(* Logix 5000 AddOnInstructionDefinition export H_ACOMM; software revision 34.01 *)

TYPE HIWIN_MIKRO_AXIS :   // HIWIN MIKROSYSTEM Servo Axis Object
STRUCT
   InData : HIWIN_MIKRO_AXIS_InData;
   OutData : HIWIN_MIKRO_AXIS_OutData;
   ConnectionFaulted : BOOL; {access Read Only}
END_STRUCT
END_TYPE

TYPE HIWIN_MIKRO_AXIS_InData :   // HIWIN MIKROSYSTEM Input Data
STRUCT
   ModesOfOperationDisplay : INT; {access Read Only}   // 6061
   Statusword : INT; {access Read Only}   // 6041
   PositionActualValue : DINT; {access Read Only}   // 6064
   VelocityActualValue : DINT; {access Read Only}   // 606C
   TorqueActualValue : INT; {access Read Only}   // 6077
   Statusword2 : HIWIN_MIKRO_Statusword2; {access None}
   FollowingErrorActualValue : DINT; {access Read Only}   // 60F4
   Rsv1 : INT; {access Read Only}   // Reserve
   DriveAlarmCode : INT; {access Read Only}
   DriveWarningCode : INT; {access Read Only}
   TouchProbeStatus : INT; {access Read Only}   // 60B9
   TouchProbe_1_PositiveEdge : DINT; {access Read Only}   // 60BA
   TouchProbe_2_PositiveEdge : DINT; {access Read Only}   // 60BA
   DigitalInput : DINT; {access Read Only}   // 60FD (bit0: P-OT, bit1: N-OT, bit16~23: I1~I8)
   Rsv2 : INT; {access Read Only}   // Reserve
   Rsv3 : INT; {access Read Only}   // Reserve
   Rsv4 : INT; {access Read Only}   // Reserve
   Rsv5 : INT; {access Read Only}   // Reserve
   UserParmMappingState : DINT; {access Read Only}   // User defined parameter mapping state
   UserMON_1 : DINT; {access Read Only}   // User defined monitor parameter 1
   UserMON_2 : DINT; {access Read Only}   // User defined monitor parameter 2
   UserMON_3 : DINT; {access Read Only}   // User defined monitor parameter 3
END_STRUCT
END_TYPE

TYPE HIWIN_MIKRO_AXIS_OutData :   // HIWIN MIKROSYSTEM Output Data
STRUCT
   ModesOfOperation : INT;   // 6060
   Controlword : INT;   // 6040
   TargetPosition : DINT;   // 607A
   TargetVelocity : DINT;   // 60FF
   TargetTorque : INT;   // 6071
   Controlword2 : INT;
   ProfileVelocity : DINT;   // 6081
   ProfileAcceleration : DINT;   // 6083
   ProfileDeceleration : DINT;   // 6084
   TorqueSlope : DINT;   // 6087
   Rsv1 : INT;   // Reserve
   TouchProbeFunction : INT;   // 60B8
   DigitalOutput : DINT;   // 60FE:01 (bit16~bit19: O1~O4)
   Rsv2 : INT;   // Reserve
   Rsv3 : INT;   // Reserve
   Rsv4 : INT;   // Reserve
   Rsv5 : INT;   // Reserve
   UserParmMappingCtrl : DINT; {access Read Only}   // User defined parameter mapping control
   UserCMD_1 : DINT;   // User defined command parameter 1
   UserCMD_2 : DINT;   // User defined command parameter 2
   UserCMD_3 : DINT;   // User defined command parameter 3
END_STRUCT
END_TYPE

TYPE HIWIN_MIKRO_Statusword2 :   // HIWIN MIKROSYSTEM Statusword2 Bit
STRUCT
   D_RDY : BOOL; {access Read Only}
   S_RDY : BOOL; {access Read Only}
   SF1 : BOOL; {access Read Only}   // STO SF1
   SF2 : BOOL; {access Read Only}   // STO SF2
   STO : BOOL; {access Read Only}   // STO
   BK : BOOL; {access Read Only}   // Brake
   CLT : BOOL; {access Read Only}   // Current Limit Active Status
   VLT : BOOL; {access Read Only}   // Velocity Limit Active Status
   COIN_VCMP : BOOL; {access Read Only}   // COIN/V_CMP Status
   NEAR : BOOL; {access Read Only}
   HOMED : BOOL; {access Read Only}
   INDEX : BOOL; {access Read Only}
   Rsv1 : BOOL; {access Read Only}
   Rsv2 : BOOL; {access Read Only}
   Rsv3 : BOOL; {access Read Only}
   Rsv4 : BOOL; {access Read Only}
END_STRUCT
END_TYPE

ADD_ON_INSTRUCTION H_ACOMM   (* revision 1.2, vendor HIWIN MIKROSYSTEM CORP., ExecutePrescan, ExecuteEnableInFalse *)
// HIWIN MIKROSYSTEM Axis Communication instruction.
// Revision note:
// Check the revision detail in Function Blocks (AOIs) Application Manual.
// Help:
// The H_ACOMM is used for drive motion and parameter IO data transmission. Each HIWIN MIKROSYSTEM axis needs a H_ACOMM instruction to create the transmission channel and remain this instruction always in enable state
VAR_IN_OUT
   InputData : INT[32]; {required}   // module:I.Data Eg. E2:I.Data
   OutputData : INT[32]; {required}   // module:O.Data Eg. E2:O.Data
   H_Axis : HIWIN_MIKRO_AXIS; {required}
END_VAR
VAR_INPUT
   ConnectionFaulted : BOOL; {required}   // 1: In connection fault state
END_VAR
VAR_OUTPUT
   EN : BOOL; {access Read Only, visible}   // 1: Instruction is enabled
   PLCControllable : BOOL; {access Read Only, visible}   // 1: Axis is controllable by PLC
   DrvErr : BOOL; {access Read Only, visible}   // 1: Drive is in alarm state
   DrvErrCode : INT; {access Read Only, visible}   // Drive error code
   DrvWarn : BOOL; {access Read Only, visible}   // 1: Drive is in warning state
   DrvWarnCode : INT; {access Read Only, visible}   // Drive warning code
   InternalLimit : BOOL; {access Read Only}   // 1: A drive internal limit is active
END_VAR
VAR
   SINT_Array : SINT[2]; {access None}
END_VAR

ROUTINE EnableInFalse   (* structured text *)
   
   // Reset output state, data
   EN := 0;
   PLCControllable := 0;
   DrvErr := 0;
   DrvWarn := 0;
   InternalLimit := 0;
   DrvErrCode := 0;
   DrvWarnCode := 0;
   
   
END_ROUTINE

ROUTINE Logic   (* structured text *)
// HIWIN MIKROSYSTEM Axis Communication
   
   //========================================
   // Update input data (drive -> controller)
   //========================================
   H_Axis.InData.ModesOfOperationDisplay	:= InputData[0];
   H_Axis.InData.Statusword				:= InputData[1];
   
   CPS(InputData[2], H_Axis.InData.PositionActualValue, 1);
   CPS(InputData[4], H_Axis.InData.VelocityActualValue, 1);
   
   H_Axis.InData.TorqueActualValue			:= InputData[6];
   
   CPS(InputData[7], H_Axis.InData.Statusword2, 1);
   CPS(InputData[8], H_Axis.InData.FollowingErrorActualValue, 1);
   
   H_Axis.InData.Rsv1 := InputData[10];
   H_Axis.InData.DriveAlarmCode			:= InputData[11];
   H_Axis.InData.DriveWarningCode			:= InputData[12];
   H_Axis.InData.TouchProbeStatus			:= InputData[13];
   
   CPS(InputData[14], H_Axis.InData.TouchProbe_1_PositiveEdge, 1);
   CPS(InputData[16], H_Axis.InData.TouchProbe_2_PositiveEdge, 1);
   CPS(InputData[18], H_Axis.InData.DigitalInput, 1);
   
   H_Axis.InData.Rsv2 := InputData[20];
   H_Axis.InData.Rsv3 := InputData[21];
   H_Axis.InData.Rsv4 := InputData[22];
   H_Axis.InData.Rsv5 := InputData[23];
   
   CPS(InputData[24], H_Axis.InData.UserParmMappingState, 1);
   CPS(InputData[26], H_Axis.InData.UserMON_1, 1);
   CPS(InputData[28], H_Axis.InData.UserMON_2, 1);
   CPS(InputData[30], H_Axis.InData.UserMON_3, 1);
   
   
   //=========================================
   // Update output data (controller -> drive)
   //=========================================
   OutputData[0] := H_Axis.OutData.ModesOfOperation;
   OutputData[1] := H_Axis.OutData.Controlword;
   
   CPS(H_Axis.OutData.TargetPosition, OutputData[2], 2);
   CPS(H_Axis.OutData.TargetVelocity, OutputData[4], 2);
   
   OutputData[6] := H_Axis.OutData.TargetTorque;
   OutputData[7] := H_Axis.OutData.Controlword2;
   
   CPS(H_Axis.OutData.ProfileVelocity, OutputData[8], 2);
   CPS(H_Axis.OutData.ProfileAcceleration, OutputData[10], 2);
   CPS(H_Axis.OutData.ProfileDeceleration, OutputData[12], 2);
   CPS(H_Axis.OutData.TorqueSlope, OutputData[14], 2);
   
   OutputData[16] := H_Axis.OutData.Rsv1;
   OutputData[17] := H_Axis.OutData.TouchProbeFunction;
   
   CPS(H_Axis.OutData.DigitalOutput, OutputData[18], 2);
   OutputData[20] := H_Axis.OutData.Rsv2;
   OutputData[21] := H_Axis.OutData.Rsv3;
   OutputData[22] := H_Axis.OutData.Rsv4;
   OutputData[23] := H_Axis.OutData.Rsv5;
   
   CPS(H_Axis.OutData.UserParmMappingCtrl, OutputData[24], 2);
   CPS(H_Axis.OutData.UserCMD_1, OutputData[26], 2);
   CPS(H_Axis.OutData.UserCMD_2, OutputData[28], 2);
   CPS(H_Axis.OutData.UserCMD_3, OutputData[30], 2);
   
   
   // Update PLCControllable state
   PLCControllable := H_Axis.InData.Statusword.9;
   
   // Update drive error state
   DrvErr := ConnectionFaulted OR H_Axis.InData.Statusword.3;
   
   // Update drive error code
   if DrvErr then
   	DrvErrCode := H_Axis.InData.DriveAlarmCode;
   else
   	DrvErrCode := 0;
   end_if;
   
   // Update drive warning state
   DrvWarn := H_Axis.InData.Statusword.7;
   
   // Update drive warning code
   if DrvWarn then
   	DrvWarnCode := H_Axis.InData.DriveWarningCode;
   else
   	DrvWarnCode := 0;
   end_if;
   
   // Update Internal Limit state
   InternalLimit := H_Axis.InData.Statusword.11;
   
   // Connection Fault
   H_Axis.ConnectionFaulted := ConnectionFaulted;
   
   // Shutdown Condition
   if (H_Axis.ConnectionFaulted
   	OR H_Axis.InData.Statusword.3
   	OR NOT PLCControllable
   	) then
   	// set Shutdown
   	H_Axis.OutData.Controlword.0 := 0;
   	H_Axis.OutData.Controlword.1 := 1;
   	H_Axis.OutData.Controlword.2 := 1;
   	H_Axis.OutData.Controlword.3 := 0;
   end_if;
   
   EN := EnableOut;
   
END_ROUTINE

ROUTINE Prescan   (* structured text *)
   // Initialize variables
   SINT_Array[0] := 0;
   SINT_Array[1] := 0;
   
   COP(SINT_Array[0] ,InputData[0], 32);
   COP(SINT_Array[0] ,OutputData[0], 32);
   
   H_Axis.InData.ModesOfOperationDisplay := 0;
   H_Axis.InData.Statusword := 0;
   H_Axis.InData.PositionActualValue := 0;
   H_Axis.InData.VelocityActualValue := 0;
   H_Axis.InData.TorqueActualValue := 0;
   COP(SINT_Array[0], H_Axis.InData.Statusword2, 1);
   H_Axis.InData.FollowingErrorActualValue := 0;
   H_Axis.InData.DigitalInput := 0;
   H_Axis.InData.DriveAlarmCode := 0;
   H_Axis.InData.DriveWarningCode := 0;
   H_Axis.InData.TouchProbeStatus := 0;
   H_Axis.InData.TouchProbe_1_PositiveEdge := 0;
   H_Axis.InData.TouchProbe_2_PositiveEdge := 0;
   H_Axis.InData.Rsv2 := 0;
   H_Axis.InData.Rsv3 := 0;
   H_Axis.InData.Rsv4 := 0;
   H_Axis.InData.Rsv5 := 0;
   H_Axis.InData.UserParmMappingState := 0;
   H_Axis.InData.UserMON_1 := 0;
   H_Axis.InData.UserMON_2 := 0;
   H_Axis.InData.UserMON_3 := 0;
   
   
   H_Axis.OutData.ModesOfOperation := 0;
   H_Axis.OutData.Controlword := 6;
   H_Axis.OutData.TargetPosition := 0;
   H_Axis.OutData.TargetVelocity := 0;
   H_Axis.OutData.TargetTorque := 0;
   H_Axis.OutData.Controlword2 := 0;
   H_Axis.OutData.ProfileVelocity := 0;
   H_Axis.OutData.ProfileAcceleration := 0;
   H_Axis.OutData.ProfileDeceleration := 0;
   H_Axis.OutData.TorqueSlope := 0;
   H_Axis.OutData.DigitalOutput := 0;
   H_Axis.OutData.TouchProbeFunction := 0;
   H_Axis.OutData.Rsv2 := 0;
   H_Axis.OutData.Rsv3 := 0;
   H_Axis.OutData.Rsv4 := 0;
   H_Axis.OutData.Rsv5 := 0;
   H_Axis.OutData.UserParmMappingCtrl := 0;
   H_Axis.OutData.UserCMD_1 := 0;
   H_Axis.OutData.UserCMD_2 := 0;
   H_Axis.OutData.UserCMD_3 := 0;
   
   H_Axis.ConnectionFaulted := 0;
   
   // Init input state, data
   ConnectionFaulted := 0;
   
   // Init output state, data
   EN := 0;
   DrvErr := 0;
   DrvWarn := 0;
   InternalLimit := 0;
   DrvErrCode := 0;
   DrvWarnCode := 0;
   
   
END_ROUTINE
END_ADD_ON_INSTRUCTION

ADD_ON_INSTRUCTION H_AStatus   (* revision 1.1, vendor HIWIN MIKROSYSTEM CORP., ExecutePrescan *)
// HIWIN MIKROSYSTEM Axis Statues instruction.
// Revision note:
// Check the revision detail in Function Blocks (AOIs) Application Manual.
VAR_IN_OUT
   H_Axis : HIWIN_MIKRO_AXIS; {required}
END_VAR
VAR_OUTPUT
   EN : BOOL; {access Read Only, visible}   // 1: Instruction is enabled
   DrvWarnCode : INT; {access Read Only, visible}   // Drive warning code
   DrvErrCode : INT; {access Read Only, visible}   // Drive error code
   D_RDY : BOOL; {access Read Only, visible}   // Drive Ready state
   S_RDY : BOOL; {access Read Only, visible}   // Servo Ready state
   DrvErr : BOOL; {access Read Only, visible}   // Drive error status
   DrvWarn : BOOL; {access Read Only, visible}   // Drive warning status
   STO : BOOL; {access Read Only, visible}   // STO active state
   SF1 : BOOL; {access Read Only, visible}   // STO SF1 input state
   SF2 : BOOL; {access Read Only, visible}   // STO SF2 input state
   BK : BOOL; {access Read Only, visible}   // Brake active state
   CLT : BOOL; {access Read Only, visible}   // Torque limit detection state
   VLT : BOOL; {access Read Only, visible}   // Velocity limit detection state
   COIN : BOOL; {access Read Only, visible}   // Positioning completion state
   V_CMP : BOOL; {access Read Only, visible}   // Velocity reach state
   NEAR : BOOL; {access Read Only, visible}   // Positioning near state
   HOMED : BOOL; {access Read Only, visible}   // Homing state
   INDEX : BOOL; {access Read Only, visible}   // Index signal output
   P_OT : BOOL; {access Read Only, visible}   // Positive limit switch
   N_OT : BOOL; {access Read Only, visible}   // Negative limit switch
   HomeSwitch : BOOL; {access Read Only, visible}   // Home switch (DOG)
   I1 : BOOL; {access Read Only, visible}   // Digital input status
   I2 : BOOL; {access Read Only, visible}   // Digital input status
   I3 : BOOL; {access Read Only, visible}   // Digital input status
   I4 : BOOL; {access Read Only, visible}   // Digital input status
   I5 : BOOL; {access Read Only, visible}   // Digital input status
   I6 : BOOL; {access Read Only, visible}   // Digital input status
   I7 : BOOL; {access Read Only, visible}   // Digital input status
   I8 : BOOL; {access Read Only, visible}   // Digital input status
END_VAR

ROUTINE Logic   (* structured text *)
// HIWIN MIKROSYSTEM Axis Servo ON
   
   D_RDY := H_Axis.InData.Statusword2.D_RDY;
   S_RDY := H_Axis.InData.Statusword2.S_RDY;
   SF1 := H_Axis.InData.Statusword2.SF1;
   SF2 := H_Axis.InData.Statusword2.SF2;
   STO := H_Axis.InData.Statusword2.STO;
   BK := H_Axis.InData.Statusword2.BK;
   CLT := H_Axis.InData.Statusword2.CLT;
   VLT := H_Axis.InData.Statusword2.VLT;
   COIN := H_Axis.InData.Statusword2.COIN_VCMP;
   V_CMP := H_Axis.InData.Statusword2.COIN_VCMP;
   NEAR := H_Axis.InData.Statusword2.NEAR;
   HOMED := H_Axis.InData.Statusword2.HOMED;
   INDEX := H_Axis.InData.Statusword2.INDEX;
   
   DrvErr := H_Axis.InData.Statusword.3;
   DrvWarn := H_Axis.InData.Statusword.7;
   
   // Update drive error code
   if DrvErr then
   	DrvErrCode := H_Axis.InData.DriveAlarmCode;
   else
   	DrvErrCode := 0;
   end_if;
   
   // Update drive warning code
   if DrvWarn then
   	DrvWarnCode := H_Axis.InData.DriveWarningCode;
   else
   	DrvWarnCode := 0;
   end_if;
   
   P_OT := H_Axis.InData.DigitalInput.0;
   N_OT := H_Axis.InData.DigitalInput.1;
   
   I1 := H_Axis.InData.DigitalInput.16;
   I2 := H_Axis.InData.DigitalInput.17;
   I3 := H_Axis.InData.DigitalInput.18;
   I4 := H_Axis.InData.DigitalInput.19;
   I5 := H_Axis.InData.DigitalInput.20;
   I6 := H_Axis.InData.DigitalInput.21;
   I7 := H_Axis.InData.DigitalInput.22;
   I8 := H_Axis.InData.DigitalInput.23;
   
END_ROUTINE

ROUTINE Prescan   (* structured text *)
   
   // Init output state, data
   EN := 0;
   
   D_RDY := 0;
   S_RDY := 0;
   SF1 := 0;
   SF2 := 0;
   STO := 0;
   BK := 0;
   CLT := 0;
   VLT := 0;
   COIN := 0;
   V_CMP := 0;
   NEAR := 0;
   HOMED := 0;
   INDEX := 0;
   
   I1 := H_Axis.InData.DigitalInput.16;
   I2 := H_Axis.InData.DigitalInput.17;
   I3 := H_Axis.InData.DigitalInput.18;
   I4 := H_Axis.InData.DigitalInput.19;
   I5 := H_Axis.InData.DigitalInput.20;
   I6 := H_Axis.InData.DigitalInput.21;
   I7 := H_Axis.InData.DigitalInput.22;
   I8 := H_Axis.InData.DigitalInput.23;
   
END_ROUTINE
END_ADD_ON_INSTRUCTION

ADD_ON_INSTRUCTION H_MAFR   (* revision 1.1, vendor HIWIN MIKROSYSTEM CORP., ExecutePrescan, ExecuteEnableInFalse *)
// HIWIN MIKROSYSTEM Axis Alarm Reset instruction.
// Revision note:
// Check the revision detail in Function Blocks (AOIs) Application Manual.
// Help:
// The H_MAFR is used to clear the drive alarms of a HIWIN MIKROSYSTEM axis.
// The command needs 20ms for execution. After 20ms, the fault reset command of Controlword will be cleared and the output of .PC will shows if drive alarms are reset successfully.
// This instruction is executed at the rising edge of enabling.
VAR_IN_OUT
   H_Axis : HIWIN_MIKRO_AXIS; {required}
END_VAR
VAR_OUTPUT
   EN : BOOL; {access Read Only, visible}   // 1: Instruction is enabled
   DN : BOOL; {access Read Only, visible}   // 1: Command execution is done
   PC : BOOL; {access None, visible}   // 1: Faults reset successfully
   IP : BOOL; {access None, visible}   // 1: Command is in processing
END_VAR
VAR
   dbOSRI : FBD_ONESHOT; {access None}
   TONR_waitToCheckState : FBD_TIMER; {access None}
   dbOSFI : FBD_ONESHOT; {access None}
END_VAR

ROUTINE EnableInFalse   (* structured text *)
   
   // Reset input
   EN := 0;
   
   // Rest OSRI func
   dbOSRI.InputBit := EnableIn;
   OSRI(dbOSRI);
   
   dbOSFI.InputBit := EnableIn;
   OSFI(dbOSFI);
   
   if dbOSFI.OutputBit then
   	TONR_waitToCheckState.PRE := 20 - TONR_waitToCheckState.ACC;
   end_if;
   
   if IP AND NOT DN then
   	TONR_waitToCheckState.TimerEnable := 1;
   	TONR(TONR_waitToCheckState);
   
   	if TONR_waitToCheckState.DN then
   		TONR_waitToCheckState.TimerEnable := 0;
   		TONR(TONR_waitToCheckState);
   		IP := 0;
   		DN := 1;
   	end_if;
   end_if;
   
   if NOT IP AND DN then
   	H_Axis.OutData.Controlword.7 := 0;
   	if NOT ((H_Axis.InData.Statusword & 16#0008) = 16#0008) then
   		PC := 1;
   	end_if;
   end_if;
   
   
   
END_ROUTINE

ROUTINE Logic   (* structured text *)
// HIWIN MIKROSYSTEM Axis Fault Reset
   // detact rising edge enable signal
   dbOSRI.InputBit := EnableIn;
   OSRI(dbOSRI);
   
   dbOSFI.InputBit := EnableIn;
   OSFI(dbOSFI);
   
   if dbOSRI.OutputBit then
   	H_Axis.OutData.Controlword.7 := 1;
   	IP := 1;
   	DN := 0;
   	PC := 0;
   end_if;
   
   if IP AND NOT DN then
   	TONR_waitToCheckState.PRE := 20; // 20ms delay
   	TONR_waitToCheckState.TimerEnable := 1;
   	TONR(TONR_waitToCheckState);
   
   	if TONR_waitToCheckState.DN then
   		TONR_waitToCheckState.TimerEnable := 0;
   		TONR(TONR_waitToCheckState);
   		IP := 0;
   		DN := 1;
   	end_if;
   end_if;
   
   if NOT IP AND DN then
   	H_Axis.OutData.Controlword.7 := 0;
   	if NOT ((H_Axis.InData.Statusword & 16#0008) = 16#0008) then
   		PC := 1;
   	end_if;
   end_if;
   
   EN := EnableOut;
   
   
END_ROUTINE

ROUTINE Prescan   (* structured text *)
   
   // Init output state, data
   EN := 0;
   DN := 0;
   
   // Init OSRI func
   dbOSRI.InputBit := 0;
   OSRI(dbOSRI);
   
   dbOSFI.InputBit := 0;
   OSFI(dbOSFI);
   
   // Reset H_Axis output data
   H_Axis.OutData.Controlword.7 := 0;
   
END_ROUTINE
END_ADD_ON_INSTRUCTION

ADD_ON_INSTRUCTION H_MAH   (* revision 1.2, vendor HIWIN MIKROSYSTEM CORP., ExecutePrescan, ExecuteEnableInFalse *)
// HIWIN MIKROSYSTEM Axis Homing instruction
// Revision note:
// Check the revision detail in Function Blocks (AOIs) Application Manual.
// Help:
// The H_MAH is used to start a CiA402 homing process on a HIWIN MIKROSYSTEM axis. The information of supported home methods is described at the drive EtherNet/IP communication command manual. (eg, E2 Series Servo Drive EtherNet_IP Communication Command Manual)
// This instruction is executed at the rising edge of enabling.
// To stop a homing process, call the H_MAS to cancel an executing command.
// [Input parameters unit]
// SearchSwitchSpeed: control unit
// SearchZeroPoint: control unit
// HomeOffset:  control unit
// [Instruction Error Codes]
// -1: PLC not controllable
// -2: Drive is in alarm state
// -3: Drive not ready
// -4: Servo not ready
// -5: Homing fail
// others: The MSG instruction error codes (referring to the Logix 5000 instruction Help file)
VAR_IN_OUT
   H_Axis : HIWIN_MIKRO_AXIS; {required}
END_VAR
VAR_INPUT
   Method : DINT; {access None, required}   // CiA402 homing method
   SearchSwitchSpeed : DINT; {access None, required}   // Calibration point (eg, a limit switch or a near home sensor) searching speed
   SearchZeroSpeed : DINT; {access None, required}   // Home point searching speed
   Acceleration : DINT; {access None, required}   // Homing acceleration
   HomeOffset : DINT; {access None, required}   // Home offset value
END_VAR
VAR_OUTPUT
   EN : BOOL; {access Read Only, visible}   // 1: Instruction is enabled
   DN : BOOL; {access Read Only, visible}   // 1: Homing process is completed or aborted
   IP : BOOL; {access Read Only, visible}   // 1: Homing process is busy
   PC : BOOL; {access Read Only, visible}   // 1: Homing is successfully completed
   ER : BOOL; {access Read Only, visible}   // 1: Instruction detect an error
   ErrCode : INT; {access Read Only, visible}   // Instruction error code
END_VAR
VAR_IN_OUT
   HomeMsgWriteCtrl : MESSAGE; {required}   // Message read/write object struct
END_VAR
VAR_INPUT
   MsgWriteData : DINT; {access None}   // DO NOT CHANGE (used to set the HomeMsgWriteCtrl 'source element')
END_VAR
VAR
   dbOSRI : FBD_ONESHOT; {access None}
   LocalStepCtrl : DINT; {access None}
   dbOSFI : FBD_ONESHOT; {access None}
   OSFI_IP : FBD_ONESHOT; {access None}
   TONR_waitToCheckState : FBD_TIMER; {access None}
END_VAR

ROUTINE EnableInFalse   (* structured text *)
   
   // Reset output state, data
   EN := 0;
   
   // Rest OSRI func
   dbOSRI.InputBit := EnableIn;
   OSRI(dbOSRI);
   
   dbOSFI.InputBit := EnableIn;
   OSFI(dbOSFI);
   
   if dbOSFI.OutputBit then
   	TONR_waitToCheckState.PRE := 50 - TONR_waitToCheckState.ACC;
   end_if;
   
   OSFI_IP.InputBit := IP;
   OSFI(OSFI_IP);
   if OSFI_IP.OutputBit then
   	H_Axis.OutData.Controlword.4 := 0;
   	OSFI_IP.InputBit := 0;
   	OSFI(OSFI_IP);
   end_if;
   
   if (LocalStepCtrl > 5) then
   
   	TONR_waitToCheckState.TimerEnable := 1;
   	TONR(TONR_waitToCheckState);
   
   	if TONR_waitToCheckState.DN then
   		if (H_Axis.InData.ModesOfOperationDisplay = 6) then
   			if H_Axis.InData.Statusword.13 then
   				// home error
   				IP := 0;
   				DN := 1;
   				ER := 1;
   				ErrCode := -5; // home fail
   				LocalStepCtrl := 0;
   
   			elsif H_Axis.InData.Statusword.10 & H_Axis.InData.Statusword.12 then
   				// home success and complete
   				IP := 0;
   				DN := 1;
   				PC := 1;
   				LocalStepCtrl := 0;
   
   			elsif H_Axis.InData.Statusword.10 & NOT H_Axis.InData.Statusword.12 & NOT H_Axis.OutData.Controlword.4 then
   				// homing process is stopped by H_MAS
   				IP := 0;
   				DN := 1;
   				PC := 0;
   				LocalStepCtrl := 0;
   
   			end_if;
   		else
   			if IP & NOT DN then
   				IP := 0;
   				DN := 1;
   				ER := 1;
   				ErrCode := -5; // home fail
   				LocalStepCtrl := 0;
   			end_if;
   		end_if;
   	end_if;
   else
   	if IP & NOT DN then
   		IP := 0;
   		DN := 1;
   		LocalStepCtrl := 0;
   	end_if;
   end_if;
   
   if NOT IP & DN then
   	TONR_waitToCheckState.TimerEnable := 0;
   	TONR(TONR_waitToCheckState);
   end_if;
   
   
   
END_ROUTINE

ROUTINE Logic   (* structured text *)
// HIWIN MIKROSYSTEM Motion Axis Homing
   
   // detact rising edge enable signal
   dbOSRI.InputBit := EnableIn;
   OSRI(dbOSRI);
   
   dbOSFI.InputBit := EnableIn;
   OSFI(dbOSFI);
   
   if dbOSRI.OutputBit then
   	IP := 1;
   	DN := 0;
   	ER := 0;
   	PC := 0;
   	ErrCode := 0;
   
   	//Request mode change
   	H_Axis.OutData.ModesOfOperation := 6; // set to Home mode
   	H_Axis.OutData.Controlword.4 := 0; // clear home start bit
   
   	LocalStepCtrl := 0;
   end_if;
   
   if IP & NOT DN then
   	if NOT H_Axis.InData.Statusword.9 then
   		IP := 0;
   		DN := 1;
   		ER := 1;
   		ErrCode := -1; // PLC not Controllable
   	elsif H_Axis.InData.Statusword.3 then
   		IP := 0;
   		DN := 1;
   		ER := 1;
   		ErrCode := -2; // Drive alarm
   	elsif NOT H_Axis.InData.Statusword2.D_RDY then
   		IP := 0;
   		DN := 1;
   		ER := 1;
   		ErrCode := -3; // Drive not ready
   	elsif NOT H_Axis.InData.Statusword2.S_RDY then
   		IP := 0;
   		DN := 1;
   		ER := 1;
   		ErrCode := -4; // Servo not ready
   	else
   		case LocalStepCtrl of
   			0: // write home method (0x6098)
   				HomeMsgWriteCtrl.Class := 16#406;
   				HomeMsgWriteCtrl.Instance := 16#098;
   				HomeMsgWriteCtrl.Attribute := 0;
   				HomeMsgWriteCtrl.REQ_LEN := 1;
   				MsgWriteData := Method;
   				MSG(HomeMsgWriteCtrl);
   
   				LocalStepCtrl := LocalStepCtrl + 1;
   
   			1: // write home acceleration (0x609A)
   				//check parameter write status
   				if NOT HomeMsgWriteCtrl.ER then
   					if HomeMsgWriteCtrl.DN then
   
   						HomeMsgWriteCtrl.Class := 16#406;
   						HomeMsgWriteCtrl.Instance := 16#09A;
   						HomeMsgWriteCtrl.Attribute := 0;
   						HomeMsgWriteCtrl.REQ_LEN := 4;
   						MsgWriteData := Acceleration;
   						MSG(HomeMsgWriteCtrl);
   
   						LocalStepCtrl := LocalStepCtrl + 1;
   					end_if;
   				else
   					IP := 0;
   					DN := 1;
   					ER := 1;
   					ErrCode := HomeMsgWriteCtrl.ERR;
   				end_if;
   
   			2: // write search switch speed (0x6099_01)
   				//check parameter write status
   				if NOT HomeMsgWriteCtrl.ER then
   					if HomeMsgWriteCtrl.DN then
   
   						HomeMsgWriteCtrl.Class := 16#406;
   						HomeMsgWriteCtrl.Instance := 16#099;
   						HomeMsgWriteCtrl.Attribute := 1;
   						HomeMsgWriteCtrl.REQ_LEN := 4;
   						MsgWriteData := SearchSwitchSpeed;
   						MSG(HomeMsgWriteCtrl);
   
   						LocalStepCtrl := LocalStepCtrl + 1;
   					end_if;
   				else
   					IP := 0;
   					DN := 1;
   					ER := 1;
   					ErrCode := HomeMsgWriteCtrl.ERR;
   				end_if;
   
   			3: // write search zero speed (0x6099_02)
   				//check parameter write status
   				if NOT HomeMsgWriteCtrl.ER then
   					if HomeMsgWriteCtrl.DN then
   
   						HomeMsgWriteCtrl.Class := 16#406;
   						HomeMsgWriteCtrl.Instance := 16#099;
   						HomeMsgWriteCtrl.Attribute := 2;
   						HomeMsgWriteCtrl.REQ_LEN := 4;
   						MsgWriteData := SearchZeroSpeed;
   						MSG(HomeMsgWriteCtrl);
   
   						LocalStepCtrl := LocalStepCtrl + 1;
   					end_if;
   				else
   					IP := 0;
   					DN := 1;
   					ER := 1;
   					ErrCode := HomeMsgWriteCtrl.ERR;
   				end_if;
   
   			4: // write home offset (0x607C)
   				//check parameter write status
   				if NOT HomeMsgWriteCtrl.ER then
   					if HomeMsgWriteCtrl.DN then
   
   						HomeMsgWriteCtrl.Class := 16#406;
   						HomeMsgWriteCtrl.Instance := 16#07C;
   						HomeMsgWriteCtrl.Attribute := 0;
   						HomeMsgWriteCtrl.REQ_LEN := 4;
   						MsgWriteData := HomeOffset;
   						MSG(HomeMsgWriteCtrl);
   
   						LocalStepCtrl := LocalStepCtrl + 1;
   					end_if;
   				else
   					IP := 0;
   					DN := 1;
   					ER := 1;
   					ErrCode := HomeMsgWriteCtrl.ERR;
   				end_if;
   
   			5:
   				//check parameter write status
   				if NOT HomeMsgWriteCtrl.ER then
   					if HomeMsgWriteCtrl.DN then
   						if (H_Axis.InData.ModesOfOperationDisplay = 6) then
   							// start homing
   							H_Axis.OutData.Controlword.4 := 1;
   							H_Axis.OutData.Controlword.8 := 0;
   
   							LocalStepCtrl := LocalStepCtrl + 1;
   						end_if;
   					end_if;
   				else
   					IP := 0;
   					DN := 1;
   					ER := 1;
   					ErrCode := HomeMsgWriteCtrl.ERR;
   				end_if;
   
   			6:
   				TONR_waitToCheckState.PRE := 50; // 50ms delay
   				TONR_waitToCheckState.TimerEnable := 1;
   				TONR(TONR_waitToCheckState);
   
   				if TONR_waitToCheckState.DN then
   					TONR_waitToCheckState.TimerEnable := 0;
   					TONR(TONR_waitToCheckState);
   					LocalStepCtrl := LocalStepCtrl + 1;
   				end_if;
   			7:
   				if (H_Axis.InData.ModesOfOperationDisplay = 6) then
   					if H_Axis.InData.Statusword.13 then
   						// home error
   						IP := 0;
   						DN := 1;
   						ER := 1;
   						ErrCode := -5; // home fail
   						LocalStepCtrl := 0;
   					elsif H_Axis.InData.Statusword.10 & H_Axis.InData.Statusword.12 then
   						// home success and complete
   						IP := 0;
   						DN := 1;
   						PC := 1;
   						LocalStepCtrl := 0;
   					elsif H_Axis.InData.Statusword.10 & NOT H_Axis.InData.Statusword.12 & NOT H_Axis.OutData.Controlword.4 then
   						// homing process is stopped by H_MAS
   						IP := 0;
   						DN := 1;
   						PC := 0;
   						LocalStepCtrl := 0;
   					end_if;
   				else
   					if IP & NOT DN then
   						IP := 0;
   						DN := 1;
   						ER := 1;
   						ErrCode := -5; // home fail
   						LocalStepCtrl := 0;
   					end_if;
   				end_if;
   		end_case;
   	end_if;
   end_if;
   
   OSFI_IP.InputBit := IP;
   OSFI(OSFI_IP);
   if OSFI_IP.OutputBit then
   	H_Axis.OutData.Controlword.4 := 0;
   	OSFI_IP.InputBit := 0;
   	OSFI(OSFI_IP);
   end_if;
   
   EN := EnableOut;
   
   
END_ROUTINE

ROUTINE Prescan   (* structured text *)
   
   // Init output state, data
   EN := 0;
   IP := 0;
   DN := 0;
   ER := 0;
   PC := 0;
   ErrCode := 0;
   
   // Init OSRI func
   dbOSRI.InputBit := 0;
   OSRI(dbOSRI);
   
   dbOSFI.InputBit := 0;
   OSFI(dbOSFI);
   
   
END_ROUTINE
END_ADD_ON_INSTRUCTION

ADD_ON_INSTRUCTION H_MAJ   (* revision 1.1, vendor HIWIN MIKROSYSTEM CORP., ExecutePrescan, ExecuteEnableInFalse *)
// HIWIN MIKROSYSTEM Axis Jog instruction
// Revision note:
// Check the revision detail in Function Blocks (AOIs) Application Manual.
// Help:
// The H_MAJ is used to an endless jogging of a HIWIN MIKROSYSTEM axis.
// This instruction is executed at the rising edge of enabling.
// A jogging can be stopped by calling H_MAS.
// [Input parameters unit]
// Speed: control unit
// Acceleration: control unit
// Deceleration:  control unit
// [Instruction Error Codes]
// -1: PLC not controllable
// -2: Drive is in alarm state
// -3: Drive not ready
// -4: Servo not ready
VAR_IN_OUT
   H_Axis : HIWIN_MIKRO_AXIS; {required}
END_VAR
VAR_INPUT
   Speed : DINT; {access None, required}   // Jogging speed
   Acceleration : DINT; {access None, required}   // Jogging acceleration
   Deceleration : DINT; {access None, required}   // Jogging deceleration
   Direction : BOOL; {access None, required}   // 0: Forward; 1: Reverse
END_VAR
VAR_OUTPUT
   EN : BOOL; {access Read Only, visible}   // 1: Instruction is enabled
   DN : BOOL; {access Read Only, visible}   // 1: Command is executed
   IP : BOOL; {access Read Only, visible}   // 0: Jogging command is stopped; 1: Jogging command is in execution
   ER : BOOL; {access Read Only, visible}   // 1: Instruction detect an error
   ErrCode : INT; {access Read Only, visible}   // Instruction error code
END_VAR
VAR
   dbOSRI : FBD_ONESHOT; {access None}
END_VAR

ROUTINE EnableInFalse   (* structured text *)
   
   // Reset output state, data
   EN := 0;
   
   // Rest OSRI func
   dbOSRI.InputBit := EnableIn;
   OSRI(dbOSRI);
   
   if NOT H_Axis.InData.Statusword2.S_RDY
   	OR NOT H_Axis.InData.Statusword2.D_RDY
   	OR H_Axis.OutData.Controlword.8  // Halt request
   	then
   	IP := 0;
   
   	H_Axis.OutData.TargetVelocity := 0;
   
   end_if;
   
END_ROUTINE

ROUTINE Logic   (* structured text *)
// HIWIN MIKROSYSTEM Axis Jog
   
   // detact rising edge enable signal
   dbOSRI.InputBit := EnableIn;
   OSRI(dbOSRI);
   
   if dbOSRI.OutputBit then
   	IP := 1;
   	DN := 0;
   	ER := 0;
   	ErrCode := 0;
   
   end_if;
   
   if IP & NOT DN then
   	if NOT H_Axis.InData.Statusword.9 then
   		ER := 1;
   		ErrCode := -1; // PLC not Controllable
   	elsif H_Axis.InData.Statusword.3 then
   		ER := 1;
   		ErrCode := -2; // Drive alarm
   	elsif NOT H_Axis.InData.Statusword2.D_RDY then
   		ER := 1;
   		ErrCode := -3; // Drive not ready
   	elsif NOT H_Axis.InData.Statusword2.S_RDY then
   		ER := 1;
   		ErrCode := -4; // Servo not ready
   	else
   		//Request mode change
   		H_Axis.OutData.ModesOfOperation := 3; // to PV
   
   	end_if;
   
   	if ER then
   		IP := 0;
   		DN := 0;
   	elsif H_Axis.InData.ModesOfOperationDisplay = 3 then
   		IP := 1;
   		DN := 1;
   
   		H_Axis.OutData.Controlword.8 := 0;
   
   		if Direction then
   			H_Axis.OutData.TargetVelocity := Speed * -1;
   		else
   			H_Axis.OutData.TargetVelocity := Speed;
   		end_if;
   		H_Axis.OutData.ProfileAcceleration := Acceleration;
   		H_Axis.OutData.ProfileDeceleration := Deceleration;
   
   	end_if;
   end_if;
   
   if IP & DN then
   	if NOT H_Axis.InData.Statusword2.S_RDY
   		OR NOT H_Axis.InData.Statusword2.D_RDY
   		OR H_Axis.OutData.Controlword.8  // Halt request
   		then
   		IP := 0;
   
   		H_Axis.OutData.TargetVelocity := 0;
   
   	end_if;
   
   end_if;
   
   EN := EnableOut;
   
   
END_ROUTINE

ROUTINE Prescan   (* structured text *)
   
   // Init output state, data
   EN := 0;
   IP := 0;
   DN := 0;
   ER := 0;
   ErrCode := 0;
   
   // Init OSRI func
   dbOSRI.InputBit := 0;
   OSRI(dbOSRI);
   
END_ROUTINE
END_ADD_ON_INSTRUCTION

ADD_ON_INSTRUCTION H_MAM   (* revision 1.1, vendor HIWIN MIKROSYSTEM CORP., ExecutePrescan, ExecuteEnableInFalse *)
// HIWIN MIKROSYSTEM Axis Positioning instruction
// Revision note:
// Check the revision detail in Function Blocks (AOIs) Application Manual.
// Help:
// The H_MAM is used to do positioning of a HIWIN MIKROSYSTEM axis. When execute the instruction every time, the setting will be active immediately.
// This instruction is executed at the rising edge of enabling.
// [Input parameters unit]
// Position: control unit
// Velocity: control unit
// Acceleration: control unit
// Deceleration:  control unit
// [Instruction Error Codes]
// -1: PLC not controllable
// -2: Drive is in alarm state
// -3: Drive not ready
// -4: Servo not ready
VAR_IN_OUT
   H_Axis : HIWIN_MIKRO_AXIS; {required}
END_VAR
VAR_INPUT
   Position : DINT; {required}   // Set position
   Velocity : DINT; {required}   // Moving velocity
   Acceleration : DINT; {required}   // Moving acceleration
   Deceleration : DINT; {required}   // Moving deceleration
   SetRelativeMove : BOOL; {required}   // 0: Move absolute; 1: Move relative
END_VAR
VAR_OUTPUT
   EN : BOOL; {access Read Only, visible}   // 1: Instruction is enabled
   DN : BOOL; {access Read Only, visible}   // 1: Command is executed
   IP : BOOL; {access Read Only, visible}   // 1: Command is in processing
   PC : BOOL; {access Read Only, visible}   // 1: Motor is in-position
   ER : BOOL; {access Read Only, visible}   // 1: Instruction detect an error
   ErrCode : INT; {access Read Only, visible}   // Instruction error code
END_VAR
VAR
   dbOSRI : FBD_ONESHOT; {access None}
   dbOSFI : FBD_ONESHOT; {access None}
END_VAR

ROUTINE EnableInFalse   (* structured text *)
   
   // Reset output state, data
   EN := 0;
   
   // Rest OSRI func
   dbOSRI.InputBit := EnableIn;
   OSRI(dbOSRI);
   
   dbOSFI.InputBit := EnableIn;
   OSFI(dbOSFI);
   
   if dbOSFI.OutputBit then
   
   	H_Axis.OutData.Controlword.4 := 0;
   	H_Axis.OutData.Controlword.5 := 0;
   
   end_if;
   
   if IP
   	& DN
   	& (H_Axis.InData.ModesOfOperationDisplay = 1)
       then
   
   	PC := H_Axis.InData.Statusword2.COIN_VCMP;
   	if PC then
   		IP := 0;
   	elsif H_Axis.OutData.Controlword.8 then
   		IP := 0;
   	end_if;
   end_if;
   
END_ROUTINE

ROUTINE Logic   (* structured text *)
// HIWIN MIKROSYSTEM Axis Positioning
   
   // detact rising edge enable signal
   dbOSRI.InputBit := EnableIn;
   OSRI(dbOSRI);
   
   dbOSFI.InputBit := EnableIn;
   OSFI(dbOSFI);
   
   if dbOSRI.OutputBit then
   	IP := 1;
   	DN := 0;
   	PC := 0;
   	ER := 0;
   	ErrCode := 0;
   
   	//Request mode change
   	H_Axis.OutData.ModesOfOperation := 1; // set to position mode
   end_if;
   
   if IP & NOT DN then
   	if NOT H_Axis.InData.Statusword.9 then
   		ER := 1;
   		ErrCode := -1; // PLC not Controllable
   	elsif H_Axis.InData.Statusword.3 then
   		ER := 1;
   		ErrCode := -2; // Drive alarm
   	elsif NOT H_Axis.InData.Statusword2.D_RDY then
   		ER := 1;
   		ErrCode := -3; // Drive not ready
   	elsif NOT H_Axis.InData.Statusword2.S_RDY then
   		ER := 1;
   		ErrCode := -4; // Servo not ready
   	else
   		if ER then
   			IP := 0;
   			DN := 0;
   		elsif H_Axis.InData.ModesOfOperationDisplay = 1 then
   
   			H_Axis.OutData.TargetPosition := Position;
   			H_Axis.OutData.Controlword.6 := SetRelativeMove;
   			H_Axis.OutData.ProfileVelocity := Velocity;
   			H_Axis.OutData.ProfileAcceleration := Acceleration;
   			H_Axis.OutData.ProfileDeceleration := Deceleration;
   
   			if NOT H_Axis.InData.Statusword.12 then
   				DN := 1;
   
   				H_Axis.OutData.Controlword.4 := 1;
   				H_Axis.OutData.Controlword.5 := 1; // change immediately
   				H_Axis.OutData.Controlword.8 := 0;
   			else
   				H_Axis.OutData.Controlword.4 := 0; // reset the new setpoint command to reset the statusword setpoint acknowledgement bit
   			end_if;
   		end_if;
   	end_if;
   end_if;
   
   if IP
   	& DN
   	& (H_Axis.InData.ModesOfOperationDisplay = 1)
       & H_Axis.InData.Statusword.12
       then
   
   	PC := H_Axis.InData.Statusword2.COIN_VCMP;
   	if PC then
   		IP := 0;
   	elsif H_Axis.OutData.Controlword.8 then
   		IP := 0;
   	end_if;
   end_if;
   
   EN := EnableOut;
   
   
END_ROUTINE

ROUTINE Prescan   (* structured text *)
   
   // Init output state, data
   EN := 0;
   IP := 0;
   DN := 0;
   PC := 0;
   ER := 0;
   ErrCode := 0;
   
   // Init OSRI func
   dbOSRI.InputBit := 0;
   OSRI(dbOSRI);
   
   dbOSFI.InputBit := 0;
   OSFI(dbOSFI);
   
   
END_ROUTINE
END_ADD_ON_INSTRUCTION

ADD_ON_INSTRUCTION H_MAR   (* revision 1.2, vendor HIWIN MIKROSYSTEM CORP., ExecutePrescan, ExecuteEnableInFalse *)
// HIWIN MIKROSYSTEM Axis Arm Registration instruction
// Revision note:
// Check the revision detail in Function Blocks (AOIs) Application Manual.
// Help:
// The H_MAR is used to arm registration event checking one time for a HIWIN MIKROSYSTEM axis. This function links to the CiA402 touch probe function of the axis.
// When the instruction is called, a registration event is armed based on the selected Registration Input (InputNumber) and the specified Trigger Condition (TriggerEdge). When the Registration Input satisfies the Trigger Condition, the motor position will be latched and stored. The latest latched position will be response at the axis input data (.InData) TouchProbe_1_PositiveEdge (word 14~15) or TouchProbe_2_PositiveEdge (word16~17).
// Use H_MDR to disarm the event checking process.
// [Instruction Error Codes]
// -1: PLC not controllable
// -6: Invalid setting value
VAR_IN_OUT
   H_Axis : HIWIN_MIKRO_AXIS; {required}
END_VAR
VAR_INPUT
   InputNumber : DINT; {access None, required}   // 0: Encoder index, 1: Ext_Probe1, 2: Ext_Probe2
   TriggerEdge : BOOL; {access None, required}   // 0: positive edge, 1: negative edge
END_VAR
VAR_OUTPUT
   EN : BOOL; {access Read Only, visible}   // 1: Instruction is enabled
   DN : BOOL; {access Read Only, visible}   // 1: Command is executed
   IP : BOOL; {access Read Only, visible}   // 1: An event checking is in processing
   PC : BOOL; {access None, visible}   // 1: A registration event occurs
   ER : BOOL; {access Read Only, visible}   // 1: Instruction detect an error
   ErrCode : INT; {access Read Only, visible}   // Instruction error code
END_VAR
VAR
   dbOSRI : FBD_ONESHOT; {access None}
   TPSignal : DINT; {access None}
   TPEdge : BOOL; {access None}
   StepCtrl : INT; {access None}   // Step control
   DrvTPStatus : INT; {access None}
END_VAR

ROUTINE EnableInFalse   (* structured text *)
   
   // Reset output state, data
   EN := 0;
   
   // Rest OSRI func
   dbOSRI.InputBit := EnableIn;
   OSRI(dbOSRI);
   
   if IP & DN & NOT ER then // waiting for the latch complete
   
   	DrvTPStatus := H_Axis.InData.TouchProbeStatus & 16#07;
   	if TPEdge then // negative edge
   		if DrvTPStatus = 16#0005 then
   			PC := 1;
   		end_if;
   	else // positive edge
   		if DrvTPStatus = 16#0003 then
   			PC := 1;
   		end_if;
   	end_if;
   
   	if ((DrvTPStatus & 16#0001) = 0) then // touch probe processing is interrupted
   		IP := 0;
   	end_if;
   
   end_if;
   
   if ER then
   	IP := 0;
   elsif IP & DN & PC then
   	IP := 0;
   elsif IP & NOT DN & StepCtrl = 2 then
   	IP := 0;
   	StepCtrl := 0;
   end_if;
   
   
   
END_ROUTINE

ROUTINE Logic   (* structured text *)
// HIWIN MIKROSYSTEM Axis Motion Arm Registration
   
   // detact rising edge enable signal
   dbOSRI.InputBit := EnableIn;
   OSRI(dbOSRI);
   
   if IP & NOT DN then
   	case StepCtrl of
   		1:
   			H_Axis.OutData.TouchProbeFunction := 16#0001;
   			StepCtrl := 2;
   		2:
   			if (H_Axis.InData.TouchProbeStatus = 16#0001) then
   				StepCtrl := 3;
   			end_if;
   		3:
   			case TPSignal of
   				0: // Encoder index
   					H_Axis.OutData.TouchProbeFunction := 16#0015;
   					DN := 1;
   					StepCtrl := 4;
   				1: // Ext_Probe 1
   					if TPEdge then // negative edge
   						H_Axis.OutData.TouchProbeFunction := 16#0021;
   					else // positive edge
   						H_Axis.OutData.TouchProbeFunction := 16#0011;
   					end_if;
   					DN := 1;
   					StepCtrl := 4;
   				else
   					ER := 1;
   					ErrCode := -6; // Invalid setting value
   			end_case;
   	end_case;
   
   elsif IP & DN then // waiting for the latch complete
   
   	DrvTPStatus := H_Axis.InData.TouchProbeStatus & 16#07;
   	if TPEdge then // negative edge
   		if DrvTPStatus = 16#0005 then
   			PC := 1;
   		end_if;
   	else // positive edge
   		if DrvTPStatus = 16#0003 then
   			PC := 1;
   		end_if;
   	end_if;
   
   	if ((DrvTPStatus & 16#0001) = 0) then
   		IP := 0;
   	end_if;
   end_if;
   
   if dbOSRI.OutputBit then
   	IP := 1;
   	DN := 0;
   	ER := 0;
   	PC := 0;
   	ErrCode := 0;
   
   	StepCtrl := 1;
   	TPSignal := InputNumber;
   	TPEdge := TriggerEdge;
   
   	if NOT H_Axis.InData.Statusword.9 then
   		IP := 0;
   		ER := 1;
   		ErrCode := -1; // PLC not controllable
   	elsif TPSignal > 3 then
   		IP := 0;
   		ER := 1;
   		ErrCode := -6; // Invalid setting value
   	end_if;
   end_if;
   
   if ER then
   	IP := 0;
   elsif IP & DN & PC then
   	IP := 0;
   end_if;
   
   EN := EnableOut;
   
   
END_ROUTINE

ROUTINE Prescan   (* structured text *)
   
   // Init output state, data
   EN := 0;
   IP := 0;
   DN := 0;
   ER := 0;
   PC := 0;
   ErrCode := 0;
   
   // Init OSRI func
   dbOSRI.InputBit := 0;
   OSRI(dbOSRI);
   
   // Init local parameters
   StepCtrl := 0;
   TPSignal := 0;
   TPEdge := 0;
   
END_ROUTINE
END_ADD_ON_INSTRUCTION

ADD_ON_INSTRUCTION H_MAS   (* revision 1.1, vendor HIWIN MIKROSYSTEM CORP., ExecutePrescan, ExecuteEnableInFalse *)
// HIWIN MIKROSYSTEM Axis Stop instruction
// Revision note:
// Check the revision detail in Function Blocks (AOIs) Application Manual.
// Help:
// The H_MAS is used to stop a moving on a HIWIN MIKROSYSTEM axis.
// The output .PC shows if the motor is stopped or not according to the setting window of PC (WindowOf_PC). The default value of the WindowOf_PC is 10. If the WindowOf_PC is not given a suitable value, the .PC state may be incorrect.
// [Input parameter unit]
// WindowOf_PC: In torque mode is 0.1% rate torque. Other modes are control unit.
// [Instruction Error Codes]
// -1: PLC not controllable
VAR_IN_OUT
   H_Axis : HIWIN_MIKRO_AXIS; {required}
END_VAR
VAR_OUTPUT
   EN : BOOL; {access Read Only, visible}   // 1: Instruction is enabled
   DN : BOOL; {access Read Only, visible}   // 1: The stop command is executed
   IP : BOOL; {access Read Only, visible}   // 1: The axis is stopping
   PC : BOOL; {access Read Only, visible}   // 1: The axis is stopped
   ER : BOOL; {access Read Only, visible}   // 1: Instruction detect an error
END_VAR
VAR_INPUT
   WindowOf_PC : DINT := 10; {required}   // The window to judge the PC true state
END_VAR
VAR_OUTPUT
   ErrCode : INT; {access Read Only, visible}   // Instruction error code
END_VAR
VAR
   dbOSRI : FBD_ONESHOT; {access None}
END_VAR

ROUTINE EnableInFalse   (* structured text *)
   
   // Reset output state, data
   EN := 0;
   
   // Rest OSRI func
   dbOSRI.InputBit := EnableIn;
   OSRI(dbOSRI);
   
   if ER then
   	IP := 0;
   end_if;
   
   if IP AND DN then
   	if (H_Axis.InData.ModesOfOperationDisplay = 4) then
   		if (ABS(H_Axis.InData.TorqueActualValue) <= WindowOf_PC) then
   			IP := 0;
   			PC := 1;
   		end_if;
   	else
   		if (ABS(H_Axis.InData.VelocityActualValue) <= WindowOf_PC) then
   			IP := 0;
   			PC := 1;
   		end_if;
   	end_if;
   end_if;
   
   
END_ROUTINE

ROUTINE Logic   (* structured text *)
// HIWIN MIKROSYSTEM Motion Axis Stop
   
   // detact rising edge enable signal
   dbOSRI.InputBit := EnableIn;
   OSRI(dbOSRI);
   
   if dbOSRI.OutputBit then
   	IP := 1;
   	DN := 0;
   	PC := 0;
   	ER := 0;
   	ErrCode := 0;
   
   end_if;
   
   if IP & NOT DN then
   	DN := 1;
   
   	if NOT H_Axis.InData.Statusword.9 then
   		IP := 0;
   		ER := 1;
   		ErrCode := -1; // PLC not Controllable
   	else
   		// set Halt to stop motion
   		H_Axis.OutData.Controlword.4 := 0;
   		H_Axis.OutData.Controlword.8 := 1;
   	end_if;
   end_if;
   
   if IP AND DN then
   	if (H_Axis.InData.ModesOfOperationDisplay = 4) then
   		if (ABS(H_Axis.InData.TorqueActualValue) <= WindowOf_PC) then
   			IP := 0;
   			PC := 1;
   		end_if;
   	else
   		if (ABS(H_Axis.InData.VelocityActualValue) <= WindowOf_PC) then
   			IP := 0;
   			PC := 1;
   		end_if;
   	end_if;
   end_if;
   
   EN := EnableOut;
   
   
END_ROUTINE

ROUTINE Prescan   (* structured text *)
   
   // Init output state, data
   EN := 0;
   IP := 0;
   DN := 0;
   PC := 0;
   ER := 0;
   ErrCode := 0;
   
   // Init OSRI func
   dbOSRI.InputBit := 0;
   OSRI(dbOSRI);
   
   
END_ROUTINE
END_ADD_ON_INSTRUCTION

ADD_ON_INSTRUCTION H_MASD   (* revision 1.1, vendor HIWIN MIKROSYSTEM CORP., ExecutePrescan, ExecuteEnableInFalse *)
// HIWIN MIKROSYSTEM Axis Shutdown instruction.
// Revision note:
// Check the revision detail in Function Blocks (AOIs) Application Manual.
// Help:
// The H_MASD is used to make a HIWIN MIKROSYSTEM axis goes into the shutdown state.
// The axis remains in the shutdown state until the H_MASR is executed.
// [Instruction Error Codes]
// -1: PLC not controllable
VAR_IN_OUT
   H_Axis : HIWIN_MIKRO_AXIS; {required}
END_VAR
VAR_OUTPUT
   EN : BOOL; {access Read Only, visible}   // 1: Instruction is enabled
   DN : BOOL; {access Read Only, visible}   // 1: Axis is shutdown successfully
   IP : BOOL; {access Read Only, visible}   // 1: Command is in processing
   ER : BOOL; {access Read Only, visible}   // 1: Instruction detect an error
   ErrCode : INT; {access Read Only, visible}   // Instruction error code
END_VAR
VAR
   dbOSRI : FBD_ONESHOT; {access None}
END_VAR

ROUTINE EnableInFalse   (* structured text *)
   
   // Reset output state, data
   EN := 0;
   
   // Rest OSRI func
   dbOSRI.InputBit := EnableIn;
   OSRI(dbOSRI);
   
   if IP then
   	// check Switch on disable state
   	if H_Axis.InData.Statusword.9 // PLCControllable
   		& NOT H_Axis.InData.Statusword.0  // not switch on
   		& NOT H_Axis.InData.Statusword.1  // not switch on
   		& NOT H_Axis.InData.Statusword.2  // not operation enable
   		& H_Axis.InData.Statusword.6  // switch on disable
   		then
   		IP := 0;
   		DN := 1;
   	end_if;
   end_if;
   
END_ROUTINE

ROUTINE Logic   (* structured text *)
// HIWIN MIKROSYSTEM Axis Shutdown
   
   // detact rising edge enable signal
   dbOSRI.InputBit := EnableIn;
   OSRI(dbOSRI);
   
   if dbOSRI.OutputBit then
   	IP := 1;
   	DN := 0;
   	ER := 0;
   	ErrCode := 0;
   end_if;
   
   if IP & NOT DN then
   	if NOT H_Axis.InData.Statusword.9 then
   		IP := 0;
   		ER := 1;
   		ErrCode := -1; // not PLCControllable
   	else
   		// set Voltage disable to goto Switch on disable state
   		H_Axis.OutData.Controlword.0 := 0;
   		H_Axis.OutData.Controlword.1 := 0;
   		H_Axis.OutData.Controlword.2 := 1;
   		H_Axis.OutData.Controlword.3 := 0;
   	end_if;
   end_if;
   
   // check Switch on disable state
   if H_Axis.InData.Statusword.9 // PLCControllable
   	& NOT H_Axis.InData.Statusword.0  // not switch on
   	& NOT H_Axis.InData.Statusword.1  // not switch on
   	& NOT H_Axis.InData.Statusword.2  // not operation enable
   	& H_Axis.InData.Statusword.6  // switch on disable
   	then
   	IP := 0;
   	DN := 1;
   end_if;
   
   EN := EnableOut;
   
   
END_ROUTINE

ROUTINE Prescan   (* structured text *)
   
   // Init output state, data
   EN := 0;
   IP := 0;
   DN := 0;
   ER := 0;
   ErrCode := 0;
   
   // Init OSRI func
   dbOSRI.InputBit := 0;
   OSRI(dbOSRI);
   
END_ROUTINE
END_ADD_ON_INSTRUCTION

ADD_ON_INSTRUCTION H_MASR   (* revision 1.1, vendor HIWIN MIKROSYSTEM CORP., ExecutePrescan, ExecuteEnableInFalse *)
// HIWIN MIKROSYSTEM Axis Shutdown Reset instruction.
// Revision note:
// Check the revision detail in Function Blocks (AOIs) Application Manual.
// Help:
// The H_MASR is used to reset a HIWIN MIKROSYSTEM axis from the shutdown state.
// [Instruction Error Codes]
// -1: PLC not controllable
VAR_IN_OUT
   H_Axis : HIWIN_MIKRO_AXIS; {required}
END_VAR
VAR_OUTPUT
   EN : BOOL; {access Read Only, visible}   // 1: Instruction is enabled
   DN : BOOL; {access Read Only, visible}   // 1: Axis is reset from the shutdown state
   IP : BOOL; {access Read Only, visible}   // 1: Command is in processing
   ER : BOOL; {access Read Only, visible}   // 1: Instruction detect an error
   ErrCode : INT; {access Read Only, visible}   // Instruction error code
END_VAR
VAR
   dbOSRI : FBD_ONESHOT; {access None}
END_VAR

ROUTINE EnableInFalse   (* structured text *)
   
   // Reset output state, data
   EN := 0;
   
   // Rest OSRI func
   dbOSRI.InputBit := EnableIn;
   OSRI(dbOSRI);
   
   if IP then
   	if H_Axis.InData.Statusword.0  // ready to switch on
   		& NOT H_Axis.InData.Statusword.1  // not switch on
   		& NOT H_Axis.InData.Statusword.2  // not operation enable
   		& H_Axis.InData.Statusword.5  // quick stop not active
   		& NOT H_Axis.InData.Statusword.6  // switch on disable
   		then
   		IP := 0;
   		DN := 1;
   	end_if;
   end_if;
   
END_ROUTINE

ROUTINE Logic   (* structured text *)
// HIWIN MIKROSYSTEM Axis Shutdown Reset
   
   // detact rising edge enable signal
   dbOSRI.InputBit := EnableIn;
   OSRI(dbOSRI);
   
   if dbOSRI.OutputBit then
   	IP := 1;
   	DN := 0;
   	ER := 0;
   	ErrCode := 0;
   end_if;
   
   if IP & NOT DN then
   	if NOT H_Axis.InData.Statusword.9 then
   		IP := 0;
   		ER := 1;
   		ErrCode := -1; // not PLCControllable
   	else
   		// set Shutdown
   		H_Axis.OutData.Controlword.0 := 0;
   		H_Axis.OutData.Controlword.1 := 1;
   		H_Axis.OutData.Controlword.2 := 1;
   		H_Axis.OutData.Controlword.3 := 0;
   	end_if;
   end_if;
   
   if IP
   	& H_Axis.InData.Statusword.0  // ready to switch on
   	& NOT H_Axis.InData.Statusword.1  // not switch on
   	& NOT H_Axis.InData.Statusword.2  // not operation enable
   	& H_Axis.InData.Statusword.5  // quick stop not active
   	& NOT H_Axis.InData.Statusword.6  // switch on disable
   	then
   	IP := 0;
   	DN := 1;
   end_if;
   
   EN := EnableOut;
   
   
END_ROUTINE

ROUTINE Prescan   (* structured text *)
   
   // Init output state, data
   EN := 0;
   IP := 0;
   DN := 0;
   ER := 0;
   ErrCode := 0;
   
   // Init OSRI func
   dbOSRI.InputBit := 0;
   OSRI(dbOSRI);
   
END_ROUTINE
END_ADD_ON_INSTRUCTION

ADD_ON_INSTRUCTION H_MAT   (* revision 1.1, vendor HIWIN MIKROSYSTEM CORP., ExecutePrescan, ExecuteEnableInFalse *)
// HIWIN MIKROSYSTEM Axis Torque instruction
// Revision note:
// Check the revision detail in Function Blocks (AOIs) Application Manual.
// Help:
// The H_MAT is used to make a torque control to a HIWIN MIKROSYSTEM axis.
// A moving by a torque control can be stopped by using H_MAS instruction,
// [Input parameters unit]
// TargetTorque: 0.1% rate torque
// TorqueOffset: 0.1% rate torque
// TorqueSlope:  0.1% rate torque
// [Instruction Error Codes]
// -1: PLC not controllable
// -2: Drive is in alarm state
// -3: Drive not ready
// -4: Servo not ready
VAR_IN_OUT
   H_Axis : HIWIN_MIKRO_AXIS; {required}
END_VAR
VAR_INPUT
   TargetTorque : INT; {access None, required}   // Target torque
   TorqueOffset : INT; {required}   // Torque offset
   TorqueSlope : INT; {access None, required}   // The rate of change of torque
END_VAR
VAR_OUTPUT
   EN : BOOL; {access Read Only, visible}   // 1: Instruction is enabled
   DN : BOOL; {access Read Only, visible}   // 1: Command is executed
   IP : BOOL; {access Read Only, visible}   // 0: Torque motion is stopped; 1: Torque motion is in execution
   ER : BOOL; {access Read Only, visible}   // 1: Instruction detect an error
   ErrCode : INT; {access Read Only, visible}   // Instruction error code
   PC : BOOL; {access Read Only}   // 1: The drive toeque is clamped at the setting torque and not reached the velocity limit
END_VAR
VAR
   dbOSRI : FBD_ONESHOT; {access None}
END_VAR

ROUTINE EnableInFalse   (* structured text *)
   
   // Reset output state, data
   EN := 0;
   
   // Rest OSRI func
   dbOSRI.InputBit := EnableIn;
   OSRI(dbOSRI);
   
   if IP & DN then
   	if NOT H_Axis.InData.Statusword2.S_RDY
   		OR NOT H_Axis.InData.Statusword2.D_RDY
   		OR H_Axis.OutData.Controlword.8  // Halt request
   		then
   		IP := 0;
   	end_if;
   
   	if (H_Axis.InData.ModesOfOperationDisplay = 4) then
   		if (H_Axis.InData.TorqueActualValue = H_Axis.OutData.TargetTorque)
   			AND NOT (H_Axis.OutData.TargetTorque = 0)
   			AND NOT H_Axis.InData.Statusword2.VLT
   			AND H_Axis.InData.Statusword.10
   			then
   			PC := 1;
   		end_if;
   	end_if;
   end_if;
   
   if NOT (H_Axis.InData.ModesOfOperationDisplay = 4) then
   	H_Axis.OutData.TargetTorque := 0;
   	IP := 0;
   	PC := 0;
   end_if;
   
END_ROUTINE

ROUTINE Logic   (* structured text *)
// HIWIN MIKROSYSTEM Motion Axis Torque
   
   // detact rising edge enable signal
   dbOSRI.InputBit := EnableIn;
   OSRI(dbOSRI);
   
   if dbOSRI.OutputBit then
   	IP := 1;
   	DN := 0;
   	PC := 0;
   	ER := 0;
   	ErrCode := 0;
   
   end_if;
   
   if IP & NOT DN then
   	if NOT H_Axis.InData.Statusword.9 then
   		ER := 1;
   		ErrCode := -1; // PLC not Controllable
   	elsif H_Axis.InData.Statusword.3 then
   		ER := 1;
   		ErrCode := -2; // Drive alarm
   	elsif NOT H_Axis.InData.Statusword2.D_RDY then
   		ER := 1;
   		ErrCode := -3; // Drive not ready
   	elsif NOT H_Axis.InData.Statusword2.S_RDY then
   		ER := 1;
   		ErrCode := -4; // Servo not ready
   	else
   		//Request mode change
   		H_Axis.OutData.ModesOfOperation := 4; // to PT
   
   	end_if;
   
   	if ER then
   		IP := 0;
   		DN := 0;
   	elsif H_Axis.InData.ModesOfOperationDisplay = 4 then
   		IP := 1;
   		DN := 1;
   
   		H_Axis.OutData.Controlword.8 := 0;
   
   		H_Axis.OutData.TargetTorque := (TargetTorque + TorqueOffset);
   		H_Axis.OutData.TorqueSlope := TorqueSlope;
   
   	end_if;
   end_if;
   
   if IP & DN then
   	if NOT H_Axis.InData.Statusword2.S_RDY
   		OR NOT H_Axis.InData.Statusword2.D_RDY
   		OR H_Axis.OutData.Controlword.8  // Halt request
   		then
   		IP := 0;
   	end_if;
   
   	if (H_Axis.InData.ModesOfOperationDisplay = 4) then
   		if (H_Axis.InData.TorqueActualValue = H_Axis.OutData.TargetTorque)
   			AND NOT (H_Axis.OutData.TargetTorque = 0)
   			AND NOT H_Axis.InData.Statusword2.VLT
   			AND H_Axis.InData.Statusword.10
   			then
   			PC := 1;
   		end_if;
   	end_if;
   end_if;
   
   if NOT (H_Axis.InData.ModesOfOperationDisplay = 4) then
   	H_Axis.OutData.TargetTorque := 0;
   	IP := 0;
   	PC := 0;
   end_if;
   
   EN := EnableOut;
   
   
END_ROUTINE

ROUTINE Prescan   (* structured text *)
   
   // Init output state, data
   EN := 0;
   IP := 0;
   DN := 0;
   PC := 0;
   ER := 0;
   ErrCode := 0;
   
   // Init OSRI func
   dbOSRI.InputBit := 0;
   OSRI(dbOSRI);
   
   
END_ROUTINE
END_ADD_ON_INSTRUCTION

ADD_ON_INSTRUCTION H_MAW   (* revision 1.1, vendor HIWIN MIKROSYSTEM CORP., ExecutePrescan, ExecuteEnableInFalse *)
// HIWIN MIKROSYSTEM Axis Arm Watch instruction
// Revision note:
// Check the revision detail in Function Blocks (AOIs) Application Manual.
// Help:
// The H_MAW is used to checking the event to a setting watch position and a trigger condition to a HIWIN MIKROSYSTEM axis.
// The PC signal will be set until both watch position and the trigger condition are fulfilling the setting.
// To disarm a watching process, use the H_MDW instruction and link it to this one.
// [Input parameters unit]
// Position: control unit
VAR_IN_OUT
   H_Axis : HIWIN_MIKRO_AXIS; {required}
END_VAR
VAR_INPUT
   Position : DINT; {access None, required}   // The watch position
   TriggerCondition : BOOL; {access None, required}   // 0: Forward direction, 1: Reverse direction
END_VAR
VAR_OUTPUT
   EN : BOOL; {access Read Only, visible}   // 1: Instruction is enabled
   DN : BOOL; {access Read Only, visible}   // 1: A watch event is armed successfully
   IP : BOOL; {access Read Only, visible}   // 1: An event is in processing
   PC : BOOL; {access None, visible}   // 1: A watch event occurs
END_VAR
VAR_INPUT
   flg_watchDisarmed : BOOL; {access None}   // DO NOT CHANGE (Used by H_MDW)
END_VAR
VAR
   dbOSRI : FBD_ONESHOT; {access None}
   watchPos : DINT; {access None}
   Direction : BOOL; {access None}
   flg_waitMovingReverse : BOOL; {access None}
END_VAR

ROUTINE EnableInFalse   (* structured text *)
   
   // Reset output state, data
   EN := 0;
   
   // Rest OSRI func
   dbOSRI.InputBit := EnableIn;
   OSRI(dbOSRI);
   
   if IP & DN then
   
   	if Direction then // reverse
   		if flg_waitMovingReverse then
   			if (H_Axis.InData.PositionActualValue > watchPos) then
   				flg_waitMovingReverse := 0;
   			end_if;
   		else
   			if (H_Axis.InData.PositionActualValue <= watchPos) then
   				PC := 1; // completely over set position
   			end_if;
   		end_if;
   	else // forward
   		if flg_waitMovingReverse then
   			if (H_Axis.InData.PositionActualValue < watchPos) then
   				flg_waitMovingReverse := 0;
   			end_if;
   		else
   			if (H_Axis.InData.PositionActualValue >= watchPos) then
   				PC := 1;
   			end_if;
   		end_if;
   	end_if;
   
   end_if;
   
   if flg_watchDisarmed then
   	IP := 0;
   elsif IP & DN then
   	if PC then
   		IP := 0;
   	end_if;
   end_if;
   
   
END_ROUTINE

ROUTINE Logic   (* structured text *)
// HIWIN MIKROSYSTEM Axis Motion Arm Watch
   
   // detact rising edge enable signal
   dbOSRI.InputBit := EnableIn;
   OSRI(dbOSRI);
   
   if IP & DN then // waiting for the position
   
   	if Direction then // reverse
   		if flg_waitMovingReverse then
   			if (H_Axis.InData.PositionActualValue > watchPos) then
   				flg_waitMovingReverse := 0;
   			end_if;
   		else
   			if (H_Axis.InData.PositionActualValue <= watchPos) then
   				PC := 1; // completely over set position
   			end_if;
   		end_if;
   	else // forward
   		if flg_waitMovingReverse then
   			if (H_Axis.InData.PositionActualValue < watchPos) then
   				flg_waitMovingReverse := 0;
   			end_if;
   		else
   			if (H_Axis.InData.PositionActualValue >= watchPos) then
   				PC := 1; // completely over set position
   			end_if;
   		end_if;
   	end_if;
   
   end_if;
   
   if dbOSRI.OutputBit then
   	flg_watchDisarmed := 0;
   	IP := 1;
   	DN := 0;
   	PC := 0;
   
   	watchPos := Position;
   	Direction := TriggerCondition;
   
   	if Direction then // reverse
   		if (H_Axis.InData.PositionActualValue < watchPos) then
   			flg_waitMovingReverse := 1;
   		else
   			flg_waitMovingReverse := 0;
   		end_if;
   	else // forward
   		if (H_Axis.InData.PositionActualValue > watchPos) then
   			flg_waitMovingReverse := 1;
   		else
   			flg_waitMovingReverse := 0;
   		end_if;
   	end_if;
   	DN := 1; // start position watching process
   end_if;
   
   if flg_watchDisarmed then
   	IP := 0;
   elsif IP & DN then
   	if PC then
   		IP := 0;
   	end_if;
   end_if;
   
   EN := EnableOut;
   
   
END_ROUTINE

ROUTINE Prescan   (* structured text *)
   
   // Init output state, data
   EN := 0;
   IP := 0;
   DN := 0;
   PC := 0;
   
   // Init OSRI func
   dbOSRI.InputBit := 0;
   OSRI(dbOSRI);
   
   // Init local parameters
   Direction := 0;
   flg_waitMovingReverse := 0;
   flg_watchDisarmed := 0;
   
   
END_ROUTINE
END_ADD_ON_INSTRUCTION

ADD_ON_INSTRUCTION H_MDW   (* revision 1.1, vendor HIWIN MIKROSYSTEM CORP., ExecutePrescan, ExecuteEnableInFalse *)
// HIWIN MIKROSYSTEM Axis Disarm Watch instruction
// Revision note:
// Check the revision detail in Function Blocks (AOIs) Application Manual.
// Help:
// The H_MDW is used to disarm a position watch event which is enabled by H_MAW of a HIWIN MIKROSYSTEM axis.
// The target H_MAW must be linked to this instruction.
VAR_IN_OUT
   H_Axis : HIWIN_MIKRO_AXIS; {required}
   Link_H_MAW : H_MAW; {required}
END_VAR
VAR_OUTPUT
   EN : BOOL; {access Read Only, visible}   // Function is enabled (same as EnableOut)
   DN : BOOL; {access Read Only, visible}
   IP : BOOL; {access Read Only, visible}
END_VAR
VAR
   dbOSRI : FBD_ONESHOT; {access None}
   watchPos : DINT; {access None}
END_VAR

ROUTINE EnableInFalse   (* structured text *)
   
   // Reset output state, data
   EN := 0;
   
   // Rest OSRI func
   dbOSRI.InputBit := EnableIn;
   OSRI(dbOSRI);
   
   if IP then
   	if NOT Link_H_MAW.IP then
   		DN := 1;
   	end_if;
   end_if;
   
   if IP & DN then
   	IP := 0;
   end_if;
   
   
END_ROUTINE

ROUTINE Logic   (* structured text *)
// HIWIN MIKROSYSTEM Axis Motion Disarm Watch
   
   // detact rising edge enable signal
   dbOSRI.InputBit := EnableIn;
   OSRI(dbOSRI);
   
   if IP then
   	if NOT Link_H_MAW.IP then
   		DN := 1;
   	end_if;
   end_if;
   
   if dbOSRI.OutputBit then
   	IP := 1;
   	DN := 0;
   
   	Link_H_MAW.flg_watchDisarmed := 1;
   
   end_if;
   
   if IP & DN then
   	IP := 0;
   end_if;
   
   EN := EnableOut;
   
   
END_ROUTINE

ROUTINE Prescan   (* structured text *)
   
   // Init output state, data
   EN := 0;
   IP := 0;
   DN := 0;
   
   // Init OSRI func
   dbOSRI.InputBit := 0;
   OSRI(dbOSRI);
   
   // Init local parameters
   
END_ROUTINE
END_ADD_ON_INSTRUCTION

ADD_ON_INSTRUCTION H_MDR   (* revision 1.1, vendor HIWIN MIKROSYSTEM CORP., ExecutePrescan, ExecuteEnableInFalse *)
// HIWIN MIKROSYSTEM Axis Disarm Registration instruction
// Revision note:
// Check the revision detail in Function Blocks (AOIs) Application Manual.
// Help:
// The H_MDR is used to disarm an armed checking event by a H_MAR of a HIWIN MIKROSYSTEM axis.
//  When the H_MDR is executed, the touch probe function enabling by H_MAR will be disabled.
// [Instruction Error Codes]
// -1: PLC not controlable
VAR_IN_OUT
   H_Axis : HIWIN_MIKRO_AXIS; {required}
END_VAR
VAR_OUTPUT
   EN : BOOL; {access Read Only, visible}   // 1: Instruction is enabled
   DN : BOOL; {access Read Only, visible}   // 1: A watch process is disarmed
   IP : BOOL; {access Read Only, visible}   // 1: Instruction is in processing
   ER : BOOL; {access Read Only, visible}   // 1: Instruction detect an error
   ErrCode : INT; {access Read Only, visible}   // Instruction error code
END_VAR
VAR
   dbOSRI : FBD_ONESHOT; {access None}
   StepCtrl : INT; {access None}   // Step control
   DrvTPStatus : INT; {access None}
END_VAR

ROUTINE EnableInFalse   (* structured text *)
   
   // Reset output state, data
   EN := 0;
   
   // Rest OSRI func
   dbOSRI.InputBit := EnableIn;
   OSRI(dbOSRI);
   
   if IP & NOT DN & NOT ER then
   	if (H_Axis.InData.TouchProbeStatus = 0) then
   		IP := 0;
   	end_if;
   end_if;
   
   if ER then
   	IP := 0;
   elsif IP & DN then
   	IP := 0;
   end_if;
   
   
   
END_ROUTINE

ROUTINE Logic   (* structured text *)
// HIWIN MIKROSYSTEM Axis Motion Disarm Registration
   
   // detact rising edge enable signal
   dbOSRI.InputBit := EnableIn;
   OSRI(dbOSRI);
   
   if dbOSRI.OutputBit then
   	IP := 1;
   	DN := 0;
   	ER := 0;
   	ErrCode := 0;
   
   	StepCtrl := 1;
   end_if;
   
   if NOT H_Axis.InData.Statusword.9 then
   	ER := 1;
   	ErrCode := -1; // PLC not controllable
   else
   	if IP & NOT DN then
   		case StepCtrl of
   			1:
   				H_Axis.OutData.TouchProbeFunction := 0;
   				StepCtrl := 2;
   			2:
   				if (H_Axis.InData.TouchProbeStatus = 0) then
   					DN := 1;
   					StepCtrl := 3;
   				end_if;
   		end_case;
   	end_if;
   end_if;
   
   if ER then
   	IP := 0;
   elsif IP & DN then
   	IP := 0;
   end_if;
   
   EN := EnableOut;
   
   
END_ROUTINE

ROUTINE Prescan   (* structured text *)
   
   // Init output state, data
   EN := 0;
   IP := 0;
   DN := 0;
   ER := 0;
   ErrCode := 0;
   
   // Init OSRI func
   dbOSRI.InputBit := 0;
   OSRI(dbOSRI);
   
   // Init local parameters
   StepCtrl := 0;
   
   
END_ROUTINE
END_ADD_ON_INSTRUCTION

ADD_ON_INSTRUCTION H_MSF   (* revision 1.1, vendor HIWIN MIKROSYSTEM CORP., ExecutePrescan, ExecuteEnableInFalse *)
// HIWIN MIKROSYSTEM Axis Servo OFF instruction
// Revision note:
// Check the revision detail in Function Blocks (AOIs) Application Manual.
// Help:
// The H_MSF is used to disable a HIWIN MIKROSYSTEM axis.
// [Instruction Error Codes]
// -1: PLC not controllable
VAR_IN_OUT
   H_Axis : HIWIN_MIKRO_AXIS; {required}
END_VAR
VAR_OUTPUT
   EN : BOOL; {access Read Only, visible}   // 1: Instruction is enabled
   DN : BOOL; {access Read Only, visible}   // 1: The axis is servo OFF successfully
   IP : BOOL; {access Read Only, visible}   // 1: A servo OFF command is in processing
   ER : BOOL; {access Read Only, visible}   // 1: Instruction detect an error
   ErrCode : INT; {access Read Only, visible}   // Instruction error code
END_VAR
VAR
   dbOSRI : FBD_ONESHOT; {access None}
END_VAR

ROUTINE EnableInFalse   (* structured text *)
   
   // Reset output state, data
   EN := 0;
   
   // Rest OSRI func
   dbOSRI.InputBit := EnableIn;
   OSRI(dbOSRI);
   
   if IP
   	& NOT H_Axis.InData.Statusword2.S_RDY // servo off
   	& NOT H_Axis.InData.Statusword.1  // not switch on
   	& NOT H_Axis.InData.Statusword.2  // not operation enable
   	then
   	IP := 0;
   	DN := 1;
   end_if;
   
END_ROUTINE

ROUTINE Logic   (* structured text *)
// HIWIN MIKROSYSTEM Axis Servo OFF
   
   // detact rising edge enable signal
   dbOSRI.InputBit := EnableIn;
   OSRI(dbOSRI);
   
   if dbOSRI.OutputBit then
   	IP := 1;
   	DN := 0;
   	ER := 0;
   	ErrCode := 0;
   end_if;
   
   if IP & NOT DN then
   	if NOT H_Axis.InData.Statusword.9 then
   		IP := 0;
   		ER := 1;
   		ErrCode := -1; // not PLCControllable
   	else
   		// set disable voltage
   		H_Axis.OutData.Controlword.0 := 0;
   		H_Axis.OutData.Controlword.1 := 1;
   		H_Axis.OutData.Controlword.2 := 1;
   		H_Axis.OutData.Controlword.3 := 0;
   	end_if;
   end_if;
   
   // check SV-OFF state
   if IP
   	& NOT H_Axis.InData.Statusword2.S_RDY // servo off
   	& NOT H_Axis.InData.Statusword.1  // not switch on
   	& NOT H_Axis.InData.Statusword.2  // not operation enable
   	then
   	IP := 0;
   	DN := 1;
   end_if;
   
   EN := EnableOut;
   
   
END_ROUTINE

ROUTINE Prescan   (* structured text *)
   
   // Init output state, data
   EN := 0;
   IP := 0;
   DN := 0;
   ER := 0;
   ErrCode := 0;
   
   // Init OSRI func
   dbOSRI.InputBit := 0;
   OSRI(dbOSRI);
   
END_ROUTINE
END_ADD_ON_INSTRUCTION

ADD_ON_INSTRUCTION H_MSO   (* revision 1.1, vendor HIWIN MIKROSYSTEM CORP., ExecutePrescan, ExecuteEnableInFalse *)
// HIWIN MIKROSYSTEM Axis Servo ON instruction.
// Revision note:
// Check the revision detail in Function Blocks (AOIs) Application Manual.
// Help:
// The H_MSO is used to servo ON a HIWIN MIKROSYSTEM axis. The servo ON process is executed by the rising edge of the H_MSO enabling.
// To disable the axis, call the H_MSF instruction.
// [Instruction Error Codes]
// -1: PLC not controllable
// -2: Drive is in alarm state
// -3: Drive not ready
VAR_IN_OUT
   H_Axis : HIWIN_MIKRO_AXIS; {required}
END_VAR
VAR_OUTPUT
   EN : BOOL; {access Read Only, visible}   // 1: Instruction is enabled
   DN : BOOL; {access Read Only, visible}   // Axis is successfully servo ON (Done)
   IP : BOOL; {access Read Only, visible}   // 1: An servo ON command is in processing
   ER : BOOL; {access Read Only, visible}   // 1: Instruction detect an error
   ErrCode : INT; {access Read Only, visible}   // Instruction error code
END_VAR
VAR
   PDS_state : INT; {access None}   // Statusword PDS bits area information
   dbOSRI : FBD_ONESHOT; {access None}
END_VAR

ROUTINE EnableInFalse   (* structured text *)
   
   // Reset output state, data
   EN := 0;
   
   // Rest OSRI func
   dbOSRI.InputBit := EnableIn;
   OSRI(dbOSRI);
   
   if IP then
   	if NOT (PDS_state = 16#0023) OR NOT (PDS_state = 16#0027) then
   		// check SV-ON state
   		if H_Axis.InData.Statusword2.S_RDY
   			& H_Axis.InData.Statusword.0  // ready to switch on
   			& H_Axis.InData.Statusword.1  // switch on
   			& H_Axis.InData.Statusword.2  // operation enable
   			then
   			IP := 0;
   			DN := 1;
   		end_if;
   	else
   		IP := 0;
   	end_if;
   end_if;
   
END_ROUTINE

ROUTINE Logic   (* structured text *)
// HIWIN MIKROSYSTEM Axis Servo ON
   
   // detact rising edge enable signal
   dbOSRI.InputBit := EnableIn;
   OSRI(dbOSRI);
   
   if dbOSRI.OutputBit then
   	IP := 1;
   	DN := 0;
   	ER := 0;
   	ErrCode := 0;
   end_if;
   
   // SV-ON process is in active
   if IP & NOT DN then
   	if NOT H_Axis.InData.Statusword.9 then
   		ER := 1;
   		ErrCode := -1; // PLC not controllable
   	elsif H_Axis.InData.Statusword.3 then
   		ER := 1;
   		ErrCode := -2; // Drive alarm
   	elsif NOT H_Axis.InData.Statusword2.D_RDY then
   		ER := 1;
   		ErrCode := -3; // Drive not ready
   	else
   		PDS_state := H_Axis.InData.Statusword AND 16#0067;
   		case PDS_state of
   			16#0040: // Switch on disable
   				// set Shutdown
   				H_Axis.OutData.Controlword.0 := 0;
   				H_Axis.OutData.Controlword.1 := 1;
   				H_Axis.OutData.Controlword.2 := 1;
   				H_Axis.OutData.Controlword.3 := 0;
   				H_Axis.OutData.Controlword.7 := 0;
   			16#0021: // Ready to switch on
   				// set Switch on
   				H_Axis.OutData.Controlword.0 := 1;
   				H_Axis.OutData.Controlword.1 := 1;
   				H_Axis.OutData.Controlword.2 := 1;
   				H_Axis.OutData.Controlword.3 := 0;
   			16#0023, 16#0027: // Switch on or Operation enable
   				// set Operation enable
   				H_Axis.OutData.Controlword.0 := 1;
   				H_Axis.OutData.Controlword.1 := 1;
   				H_Axis.OutData.Controlword.2 := 1;
   				H_Axis.OutData.Controlword.3 := 1;
   			else
   				// Invalid PDS state
   				ER := 1;
   				ErrCode := -10;
   		end_case;
   	end_if;
   
   	if ER then
   		IP := 0;
   		// set Shutdown
   		H_Axis.OutData.Controlword.0 := 0;
   		H_Axis.OutData.Controlword.1 := 1;
   		H_Axis.OutData.Controlword.2 := 1;
   		H_Axis.OutData.Controlword.3 := 0;
   	end_if;
   end_if;
   
   // check SV-ON state
   if IP
   	& H_Axis.InData.Statusword2.S_RDY
   	& H_Axis.InData.Statusword.0  // ready to switch on
   	& H_Axis.InData.Statusword.1  // switch on
   	& H_Axis.InData.Statusword.2  // operation enable
   	then
   	IP := 0;
   	DN := 1;
   end_if;
   
   EN := EnableOut;
   
   
END_ROUTINE

ROUTINE Prescan   (* structured text *)
   
   // Init output state, data
   EN := 0;
   IP := 0;
   DN := 0;
   ER := 0;
   ErrCode := 0;
   
   PDS_state := 0;
   
   // Init OSRI func
   dbOSRI.InputBit := 0;
   OSRI(dbOSRI);
   
END_ROUTINE
END_ADD_ON_INSTRUCTION

ADD_ON_INSTRUCTION H_ParmRead_Single   (* revision 1.1, vendor HIWIN MIKROSYSTEM CORP., ExecutePrescan, ExecuteEnableInFalse *)
// Read a HIWIN MIKROSYSTEM Axis Parameter
// Revision note:
// Check the revision detail in Function Blocks (AOIs) Application Manual.
// Help:
// The H_ParmRead_Single is used to read a parameter of a HIWIN MIKROSYSTEM axis. When the function is called, it will start an MSG read process one time.
// The instruction is rising edge enabling. See the drive communication command manual for a parameter NO and the subindex. If the flag of Is_Data_REAL is set, the data receives from an axis will be considered as a REAL type and displayed at the ReadValue_REAL output. Otherwise, the data receives from an axis will be considered as an integer type and displayed at the ReadValue output.
// The MSG_ErrCode and MSG_ExtErrCode display the error code and the extension error code of the MSG instruction of the Logix 5000.
// [Input parameters unit]
// Parm_NO: The hex value of the object number of the target parameter
// Parm_SubIndex: The hex value of the subindex of the target parameter
VAR_IN_OUT
   H_Axis : HIWIN_MIKRO_AXIS; {required}
END_VAR
VAR_INPUT
   Parm_NO : INT; {required}   // Parameter NO
   Parm_Subindex : SINT; {access None, required}   // Parameter subindex
   Is_Data_REAL : BOOL; {required}   // 0: Read data as the integer type; 1: Read data as the REAL type
END_VAR
VAR_OUTPUT
   ReadValue : DINT; {access Read Only, required}   // An integer output of the read value
   ReadValue_REAL : REAL; {access Read Only, required}   // A REAL output of the read value
   EN : BOOL; {access Read Only, visible}   // 1: Instruction is enabled
   DN : BOOL; {access Read Only, visible}   // 1: Reading process is completed or error
   IP : BOOL; {access Read Only, visible}   // 1: A reading request is in processing
   ER : BOOL; {access Read Only, visible}   // 1: Instruction detect an error
END_VAR
VAR_IN_OUT
   MSG_Read : MESSAGE; {required}
END_VAR
VAR_OUTPUT
   MSG_ErrCode : INT; {access Read Only, visible}   // MSG error code
   MSG_ExtErrCode : DINT; {access Read Only, visible}   // MSG extended error codes
END_VAR
VAR_INPUT
   MsgReadData : DINT; {access None}   // DO NOT CHANGE (Used for MSG setting window)
END_VAR
VAR
   MSG_ERR : INT; {access None}
   dbOSRI : FBD_ONESHOT; {access None}
   dbOSFI : FBD_ONESHOT; {access None}
   MSG_ST_status : BOOL; {access None}
   MSG_DN_status : BOOL; {access None}
   MSG_ER_status : BOOL; {access None}
   MSG_EXERR : DINT; {access None}
END_VAR

ROUTINE EnableInFalse   (* structured text *)
   
   // Reset output state, data
   EN := 0;
   
   // Rest OSRI func
   dbOSRI.InputBit := EnableIn;
   OSRI(dbOSRI);
   
   dbOSFI.InputBit := EnableIn;
   OSFI(dbOSFI);
   
   MSG_ST_status := MSG_Read.ST;
   MSG_DN_status := MSG_Read.DN;
   MSG_ER_status := MSG_Read.ER;
   MSG_ERR := MSG_Read.ERR;
   MSG_EXERR := MSG_Read.EXERR;
   
   if NOT MSG_ST_status & MSG_DN_status then
   	IP := 0;
   	DN := 1;
   
   	if Is_Data_REAL then
   		CPS(MsgReadData, ReadValue_REAL, 1);
   	else
   		CPS(MsgReadData, ReadValue, 1);
   	end_if;
   
   elsif MSG_ER_status then
   	IP := 0;
   	ER := 1;
   
   	MSG_ErrCode := MSG_ERR;
   	MSG_ExtErrCode := MSG_EXERR;
   end_if;
   
   
END_ROUTINE

ROUTINE Logic   (* structured text *)
// Read a HIWIN MIKROSYSTEM axis parameter
   // detact rising edge enable signal
   dbOSRI.InputBit := EnableIn;
   OSRI(dbOSRI);
   
   dbOSFI.InputBit := EnableIn;
   OSFI(dbOSFI);
   
   if dbOSRI.OutputBit then // new process active
   	IP := 1;
   	DN := 0;
   	ER := 0;
   	MSG_ErrCode := 0;
   	MSG_ExtErrCode := 0;
   
   	MSG_ST_status := 0;
   	MSG_DN_status := 0;
   	MSG_ER_status := 0;
   	MSG_ERR := 0;
   	MSG_EXERR := 0;
   
   	ReadValue := 0;
   	ReadValue_REAL := 0;
   	MsgReadData := 0;
   end_if;
   
   
   if IP & NOT DN then // new command in process
   	case (Parm_NO & 16#F000) of
   		16#2000, 16#3000, 16#4000:
   			MSG_Read.Class := 16#405;
   			MSG_Read.Instance := 1;
   			MSG_Read.Attribute := Parm_NO;
   
   		16#6000:
   			MSG_Read.Class := 16#406;
   			MSG_Read.Instance := (Parm_NO & 16#0FFF);
   			MSG_Read.Attribute := Parm_Subindex;
   
   	end_case;
   
   	MSG(MSG_Read);
   
   	MSG_ST_status := MSG_Read.ST;
   	MSG_DN_status := MSG_Read.DN;
   	MSG_ER_status := MSG_Read.ER;
   	MSG_ERR := MSG_Read.ERR;
   	MSG_EXERR := MSG_Read.EXERR;
   
   	if NOT MSG_ST_status & MSG_DN_status then
   		IP := 0;
   		DN := 1;
   
   		if Is_Data_REAL then
   			CPS(MsgReadData, ReadValue_REAL, 1);
   		else
   			CPS(MsgReadData, ReadValue, 1);
   		end_if;
   
   	elsif MSG_ER_status then
   		IP := 0;
   		ER := 1;
   
   		MSG_ErrCode := MSG_ERR;
   		MSG_ExtErrCode := MSG_EXERR;
   	end_if;
   
   end_if;
   
   EN := EnableOut;
   
   
   
END_ROUTINE

ROUTINE Prescan   (* structured text *)
   // Init output state, data
   EN := 0;
   IP := 0;
   DN := 0;
   ER := 0;
   MSG_ErrCode := 0;
   MSG_ExtErrCode := 0;
   
   MSG_ST_status := 0;
   MSG_DN_status := 0;
   MSG_ER_status := 0;
   MSG_ERR := 0;
   MSG_EXERR := 0;
   
   // Init OSRI func
   dbOSRI.InputBit := 0;
   OSRI(dbOSRI);
   dbOSFI.InputBit := 1;
   OSFI(dbOSFI);
   
   // Init local data
   // N/A
   
   
END_ROUTINE
END_ADD_ON_INSTRUCTION

ADD_ON_INSTRUCTION H_ParmWrite_Single   (* revision 1.2, vendor HIWIN MIKROSYSTEM CORP., ExecutePrescan, ExecuteEnableInFalse *)
// Write a HIWIN MIKROSYSTEM Axis Parameter
// Revision note:
// Check the revision detail in Function Blocks (AOIs) Application Manual.
// Help:
// The H_ParmRead_Single is used to write a parameter of a HIWIN MIKROSYSTEM axis. When the function is called, it will start an MSG write process one time.
// The instruction is rising edge enabling. See the drive communication command manual for a parameter NO and the subindex. If the flag of Is_Data_REAL is set, the instruction will use the WriteValue_REAL as the input sourceto send to the axis. Otherwise, the WriteValue will be used as the input source to send to the axis. The Data_Length must be set correctly according to the parameter data type. Otherwise, an error will occur.
// The MSG_ErrCode and MSG_ExtErrCode display the error code and the extension error code of the MSG instruction of the Logix 5000.
// [Input parameters]
// Parm_NO: The hex value of the object number of the target parameter
// Parm_SubIndex: The hex value of the subindex of the target parameter
// Data_Length: byte
VAR_IN_OUT
   H_Axis : HIWIN_MIKRO_AXIS; {required}
END_VAR
VAR_INPUT
   Parm_NO : INT; {required}   // Parameter NO
   Parm_Subindex : SINT; {access None, required}   // Parameter subindex
   Data_Length : INT; {access Read Only, required}   // Parameter data length
   Is_Data_REAL : BOOL; {required}   // 0: Write data from the WriteValue; 1: Write data from the WriteValue_REAL
   WriteValue : DINT; {required}   // The integer writing value
   WriteValue_REAL : REAL; {required}   // The REAL writinge value
END_VAR
VAR_OUTPUT
   EN : BOOL; {access Read Only, visible}   // 1: Instruction is enabled
   DN : BOOL; {access Read Only, visible}   // 1: Writing process is completed or error
   IP : BOOL; {access Read Only, visible}   // 1: A writing request is in processing
   ER : BOOL; {access Read Only, visible}   // 1: Instruction detect an error
END_VAR
VAR_IN_OUT
   MSG_Write : MESSAGE; {required}
END_VAR
VAR_OUTPUT
   MSG_ErrCode : INT; {access Read Only, visible}   // MSG error code
   MSG_ExtErrCode : DINT; {access Read Only, visible}   // MSG extended error codes
END_VAR
VAR_INPUT
   MsgWriteData : DINT;   // DO NOT CHANGE (Used for MSG setting window)
END_VAR
VAR
   MSG_ERR : INT; {access None}
   dbOSRI : FBD_ONESHOT; {access None}
   dbOSFI : FBD_ONESHOT; {access None}
   MSG_ST_status : BOOL; {access None}
   MSG_DN_status : BOOL; {access None}
   MSG_ER_status : BOOL; {access None}
   MSG_EXERR : DINT; {access None}
END_VAR

ROUTINE EnableInFalse   (* structured text *)
   
   // Reset output state, data
   EN := 0;
   
   // Rest OSRI func
   dbOSRI.InputBit := EnableIn;
   OSRI(dbOSRI);
   
   dbOSFI.InputBit := EnableIn;
   OSFI(dbOSFI);
   
   MSG_ST_status := MSG_Write.ST;
   MSG_DN_status := MSG_Write.DN;
   MSG_ER_status := MSG_Write.ER;
   MSG_ERR := MSG_Write.ERR;
   MSG_EXERR := MSG_Write.EXERR;
   
   if NOT MSG_ST_status & MSG_DN_status then
   	IP := 0;
   	DN := 1;
   elsif MSG_ER_status then
   	IP := 0;
   	ER := 1;
   
   	MSG_ErrCode := MSG_ERR;
   	MSG_ExtErrCode := MSG_EXERR;
   end_if;
   
   
END_ROUTINE

ROUTINE Logic   (* structured text *)
// Write a HIWIN MIKROSYSTEM axis parameter
   // detact rising edge enable signal
   dbOSRI.InputBit := EnableIn;
   OSRI(dbOSRI);
   
   dbOSFI.InputBit := EnableIn;
   OSFI(dbOSFI);
   
   if dbOSRI.OutputBit then // new process active
   	IP := 1;
   	DN := 0;
   	ER := 0;
   	MSG_ErrCode := 0;
   	MSG_ExtErrCode := 0;
   
   	MSG_ST_status := 0;
   	MSG_DN_status := 0;
   	MSG_ER_status := 0;
   	MSG_ERR := 0;
   	MSG_EXERR := 0;
   	MsgWriteData := 0;
   end_if;
   
   if IP & NOT DN then // new command in process
   
   	if Is_Data_REAL then
   		CPS(WriteValue_REAL, MsgWriteData, 1);
   	else
   		CPS(WriteValue, MsgWriteData, 1);
   	end_if;
   
   	case (Parm_NO & 16#F000) of
   		16#2000, 16#3000, 16#4000:
   			MSG_Write.Class := 16#405;
   			MSG_Write.Instance := 1;
   			MSG_Write.Attribute := Parm_NO;
   
   		16#6000:
   			MSG_Write.Class := 16#406;
   			MSG_Write.Instance := (Parm_NO & 16#0FFF);
   			MSG_Write.Attribute := Parm_Subindex;
   
   	end_case;
   
   	MSG_Write.REQ_LEN := Data_Length;
   
   	MSG(MSG_Write);
   
   	MSG_ST_status := MSG_Write.ST;
   	MSG_DN_status := MSG_Write.DN;
   	MSG_ER_status := MSG_Write.ER;
   	MSG_ERR := MSG_Write.ERR;
   	MSG_EXERR := MSG_Write.EXERR;
   
   	if NOT MSG_ST_status & MSG_DN_status then
   		IP := 0;
   		DN := 1;
   	elsif MSG_ER_status then
   		IP := 0;
   		ER := 1;
   
   		MSG_ErrCode := MSG_ERR;
   		MSG_ExtErrCode := MSG_EXERR;
   	end_if;
   end_if;
   
   EN := EnableOut;
   
   
   
END_ROUTINE

ROUTINE Prescan   (* structured text *)
   // Init output state, data
   EN := 0;
   IP := 0;
   DN := 0;
   ER := 0;
   MSG_ErrCode := 0;
   MSG_ExtErrCode := 0;
   
   MSG_ST_status := 0;
   MSG_DN_status := 0;
   MSG_ER_status := 0;
   MSG_ERR := 0;
   MSG_EXERR := 0;
   
   // Init OSRI func
   dbOSRI.InputBit := 0;
   OSRI(dbOSRI);
   dbOSFI.InputBit := 1;
   OSFI(dbOSFI);
   
   // Init local data
   // N/A
   
   
END_ROUTINE
END_ADD_ON_INSTRUCTION
